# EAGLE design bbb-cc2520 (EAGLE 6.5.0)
AUTHOR: Neal Jackson; REV: D; TITLE: GAP

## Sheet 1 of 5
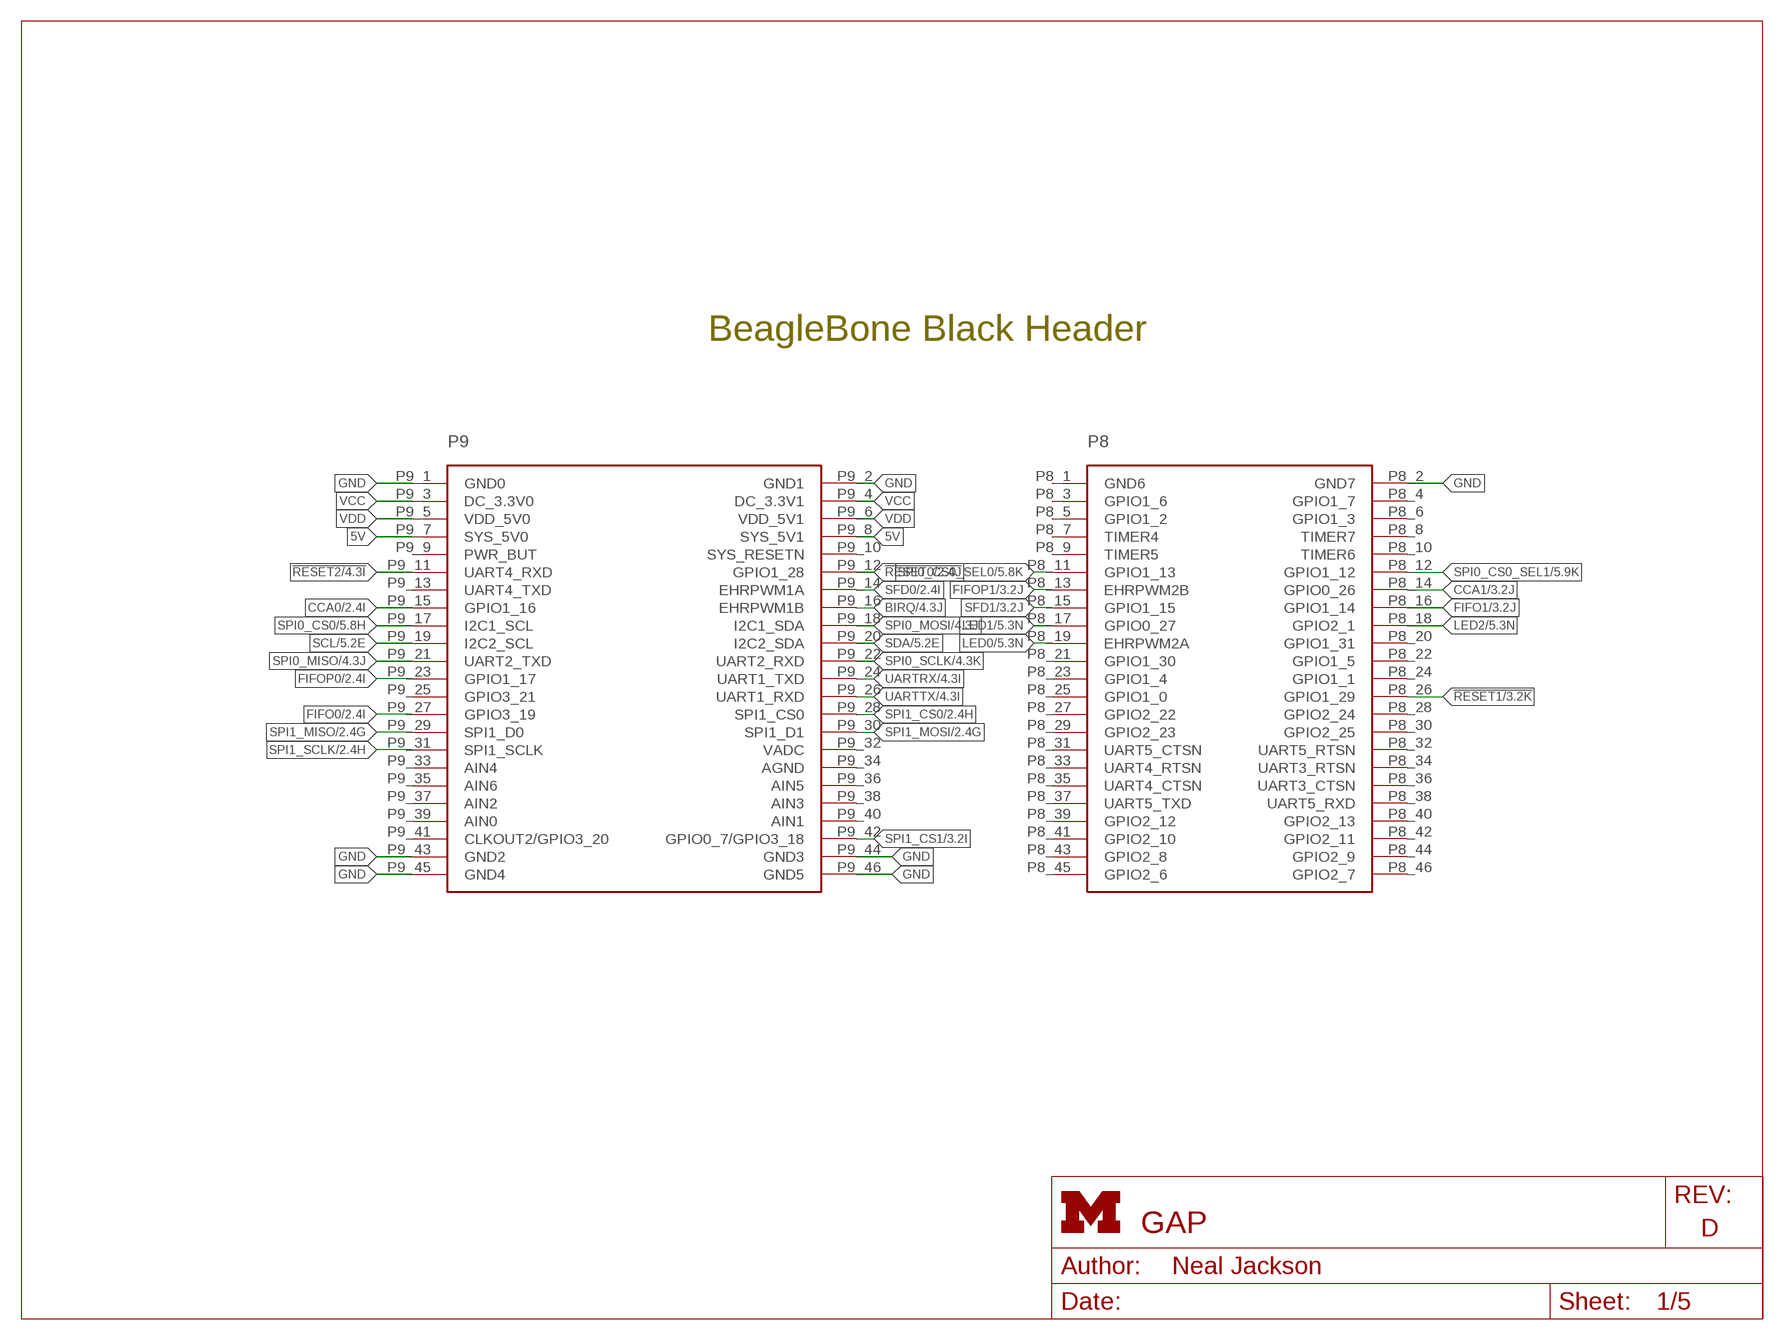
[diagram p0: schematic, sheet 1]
FRAME1 (LETTER_L): HEIGHT: 8.5in; WIDTH: 11in

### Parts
P9/P8  BBB_HEADERS  [BBB_HEADERS]

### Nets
5V: P9/P8.P9_7(SYS_5V0) P9/P8.P9_8(SYS_5V1)
!RESET0: P9/P8.P9_12(GPIO1_28) ; also sheet 2
!RESET1: P9/P8.P8_26(GPIO1_29) ; also sheet 3
!RESET2: P9/P8.P9_11(UART4_RXD) ; also sheet 4
BIRQ: P9/P8.P9_16(EHRPWM1B) ; also sheet 4
CCA0: P9/P8.P9_15(GPIO1_16) ; also sheet 2
CCA1: P9/P8.P8_14(GPIO0_26) ; also sheet 3
FIFO0: P9/P8.P9_27(GPIO3_19) ; also sheet 2
FIFO1: P9/P8.P8_16(GPIO1_14) ; also sheet 3
FIFOP0: P9/P8.P9_23(GPIO1_17) ; also sheet 2
FIFOP1: P9/P8.P8_13(EHRPWM2B) ; also sheet 3
GND: P9/P8.P8_2(GND7) P9/P8.P9_1(GND0) P9/P8.P9_2(GND1) P9/P8.P9_43(GND2) P9/P8.P9_44(GND3) P9/P8.P9_45(GND4) P9/P8.P9_46(GND5) ; also sheet 2,3,4,5
LED0: P9/P8.P8_19(EHRPWM2A) ; also sheet 5
LED1: P9/P8.P8_17(GPIO0_27) ; also sheet 5
LED2: P9/P8.P8_18(GPIO2_1) ; also sheet 5
SCL: P9/P8.P9_19(I2C2_SCL) ; also sheet 5
SDA: P9/P8.P9_20(I2C2_SDA) ; also sheet 5
SFD0: P9/P8.P9_14(EHRPWM1A) ; also sheet 2
SFD1: P9/P8.P8_15(GPIO1_15) ; also sheet 3
SPI0_CS0: P9/P8.P9_17(I2C1_SCL) ; also sheet 5
SPI0_CS0_SEL0: P9/P8.P8_11(GPIO1_13) ; also sheet 5
SPI0_CS0_SEL1: P9/P8.P8_12(GPIO1_12) ; also sheet 5
SPI0_MISO: P9/P8.P9_21(UART2_TXD) ; also sheet 4
SPI0_MOSI: P9/P8.P9_18(I2C1_SDA) ; also sheet 4
SPI0_SCLK: P9/P8.P9_22(UART2_RXD) ; also sheet 4
SPI1_CS0: P9/P8.P9_28(SPI1_CS0) ; also sheet 2
SPI1_CS1: P9/P8.P9_42(GPIO0_7/GPIO3_18) ; also sheet 3
SPI1_MISO: P9/P8.P9_29(SPI1_D0) ; also sheet 2,3
SPI1_MOSI: P9/P8.P9_30(SPI1_D1) ; also sheet 2,3
SPI1_SCLK: P9/P8.P9_31(SPI1_SCLK) ; also sheet 2,3
UARTRX: P9/P8.P9_24(UART1_TXD) ; also sheet 4
UARTTX: P9/P8.P9_26(UART1_RXD) ; also sheet 4
VCC: P9/P8.P9_3(DC_3.3V0) P9/P8.P9_4(DC_3.3V1) ; also sheet 2,3,4,5
VDD: P9/P8.P9_5(VDD_5V0) P9/P8.P9_6(VDD_5V1)
Unconnected: P9/P8.P8_1(GND6) P9/P8.P8_3(GPIO1_6) P9/P8.P8_4(GPIO1_7) P9/P8.P8_5(GPIO1_2) P9/P8.P8_6(GPIO1_3) P9/P8.P8_7(TIMER4) P9/P8.P8_8(TIMER7) P9/P8.P8_9(TIMER5) P9/P8.P8_10(TIMER6) P9/P8.P8_20(GPIO1_31) P9/P8.P8_21(GPIO1_30) P9/P8.P8_22(GPIO1_5) P9/P8.P8_23(GPIO1_4) P9/P8.P8_24(GPIO1_1) P9/P8.P8_25(GPIO1_0) P9/P8.P8_27(GPIO2_22) P9/P8.P8_28(GPIO2_24) P9/P8.P8_29(GPIO2_23) P9/P8.P8_30(GPIO2_25) P9/P8.P8_31(UART5_CTSN) P9/P8.P8_32(UART5_RTSN) P9/P8.P8_33(UART4_RTSN) P9/P8.P8_34(UART3_RTSN) P9/P8.P8_35(UART4_CTSN) P9/P8.P8_36(UART3_CTSN) P9/P8.P8_37(UART5_TXD) P9/P8.P8_38(UART5_RXD) P9/P8.P8_39(GPIO2_12) P9/P8.P8_40(GPIO2_13) P9/P8.P8_41(GPIO2_10) P9/P8.P8_42(GPIO2_11) P9/P8.P8_43(GPIO2_8) P9/P8.P8_44(GPIO2_9) P9/P8.P8_45(GPIO2_6) P9/P8.P8_46(GPIO2_7) P9/P8.P9_9(PWR_BUT) P9/P8.P9_10(SYS_RESETN) P9/P8.P9_13(UART4_TXD) P9/P8.P9_25(GPIO3_21) P9/P8.P9_32(VADC) P9/P8.P9_33(AIN4) P9/P8.P9_34(AGND) P9/P8.P9_35(AIN6) P9/P8.P9_36(AIN5) P9/P8.P9_37(AIN2) P9/P8.P9_38(AIN3) P9/P8.P9_39(AIN0) P9/P8.P9_40(AIN1) P9/P8.P9_41(CLKOUT2/GPIO3_20)

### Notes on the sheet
- BeagleBone Black Header

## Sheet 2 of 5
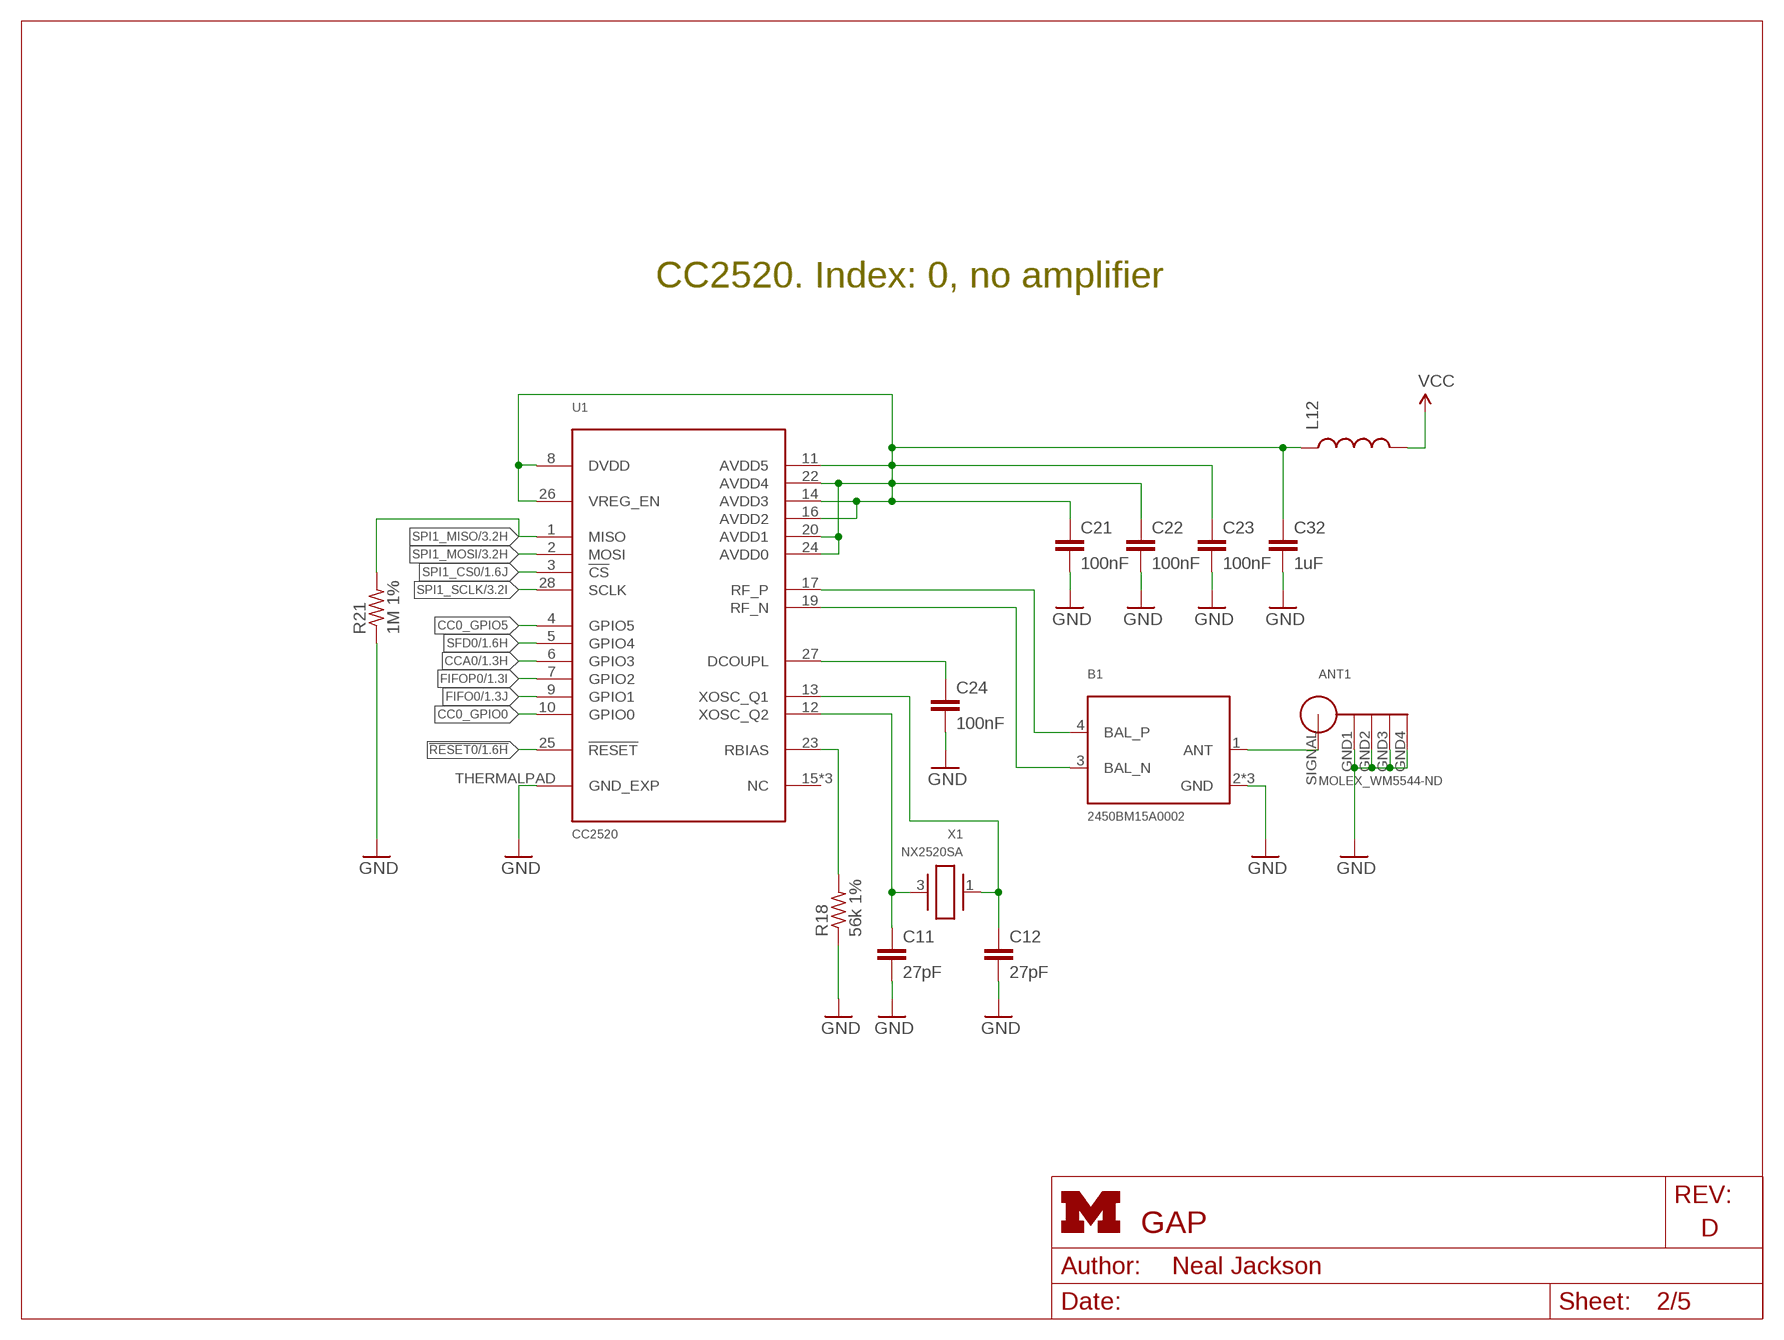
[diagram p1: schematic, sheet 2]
FRAME6 (LETTER_L): HEIGHT: 8.5in; WIDTH: 11in

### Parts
ANT1  MOLEX_WM5544-ND  [MOLEX_WM5544-ND]
B1  2450BM15A0002  [2450BM]
C11  27pF  C-EUC0402  [C0402]
C12  27pF  C-EUC0402  [C0402]
C21  100nF  C-EUC0402  [C0402]
C22  100nF  C-EUC0402  [C0402]
C23  100nF  C-EUC0402  [C0402]
C24  100nF  C-EUC0402  [C0402]
C32  1uF  C-EUC0603  [C0603]
L12  INDUCTOR0603  [0603]
R18  56k 1%  R-US_R0402  [R0402]
R21  1M 1%  R-US_R0402  [R0402]
U1  CC2520  [S-PVQFN-N28]
X1  NX2520SA  [NX2520SA]

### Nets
!RESET0: U1.25(!RESET) ; also sheet 1
CC0_GPIO0: U1.10(GPIO0)
CC0_GPIO5: U1.4(GPIO5)
CCA0: U1.6(GPIO3) ; also sheet 1
FIFO0: U1.9(GPIO1) ; also sheet 1
FIFOP0: U1.7(GPIO2) ; also sheet 1
GND: ANT1.GND1 ANT1.GND2 ANT1.GND3 ANT1.GND4 B1.2(GND) B1.5(GND) B1.6(GND) C11.2 C12.2 C21.2 C22.2 C23.2 C24.2 C32.2 R18.1 R21.1 U1.THERMALPAD(GND_EXP) ; also sheet 1,3,4,5
N$5: C21.1 C22.1 C23.1 C32.1 L12.1 U1.8(DVDD) U1.11(AVDD5) U1.14(AVDD3) U1.16(AVDD2) U1.20(AVDD1) U1.22(AVDD4) U1.24(AVDD0) U1.26(VREG_EN)
N$7: ANT1.SIGNAL B1.1(ANT)
N$11: C12.1 U1.13(XOSC_Q1) X1.1
N$12: C24.1 U1.27(DCOUPL)
N$13: C11.1 U1.12(XOSC_Q2) X1.3
N$14: R18.2 U1.23(RBIAS)
RF_N: B1.3(BAL_N) U1.19(RF_N)
RF_P: B1.4(BAL_P) U1.17(RF_P)
SFD0: U1.5(GPIO4) ; also sheet 1
SPI1_CS0: U1.3(!CS) ; also sheet 1
SPI1_MISO: R21.2 U1.1(MISO) ; also sheet 1,3
SPI1_MOSI: U1.2(MOSI) ; also sheet 1,3
SPI1_SCLK: U1.28(SCLK) ; also sheet 1,3
VCC: L12.2 ; also sheet 1,3,4,5
Unconnected: U1.15(NC) U1.18(NC) U1.21(NC)

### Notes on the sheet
- CC2520. Index: 0, no amplifier

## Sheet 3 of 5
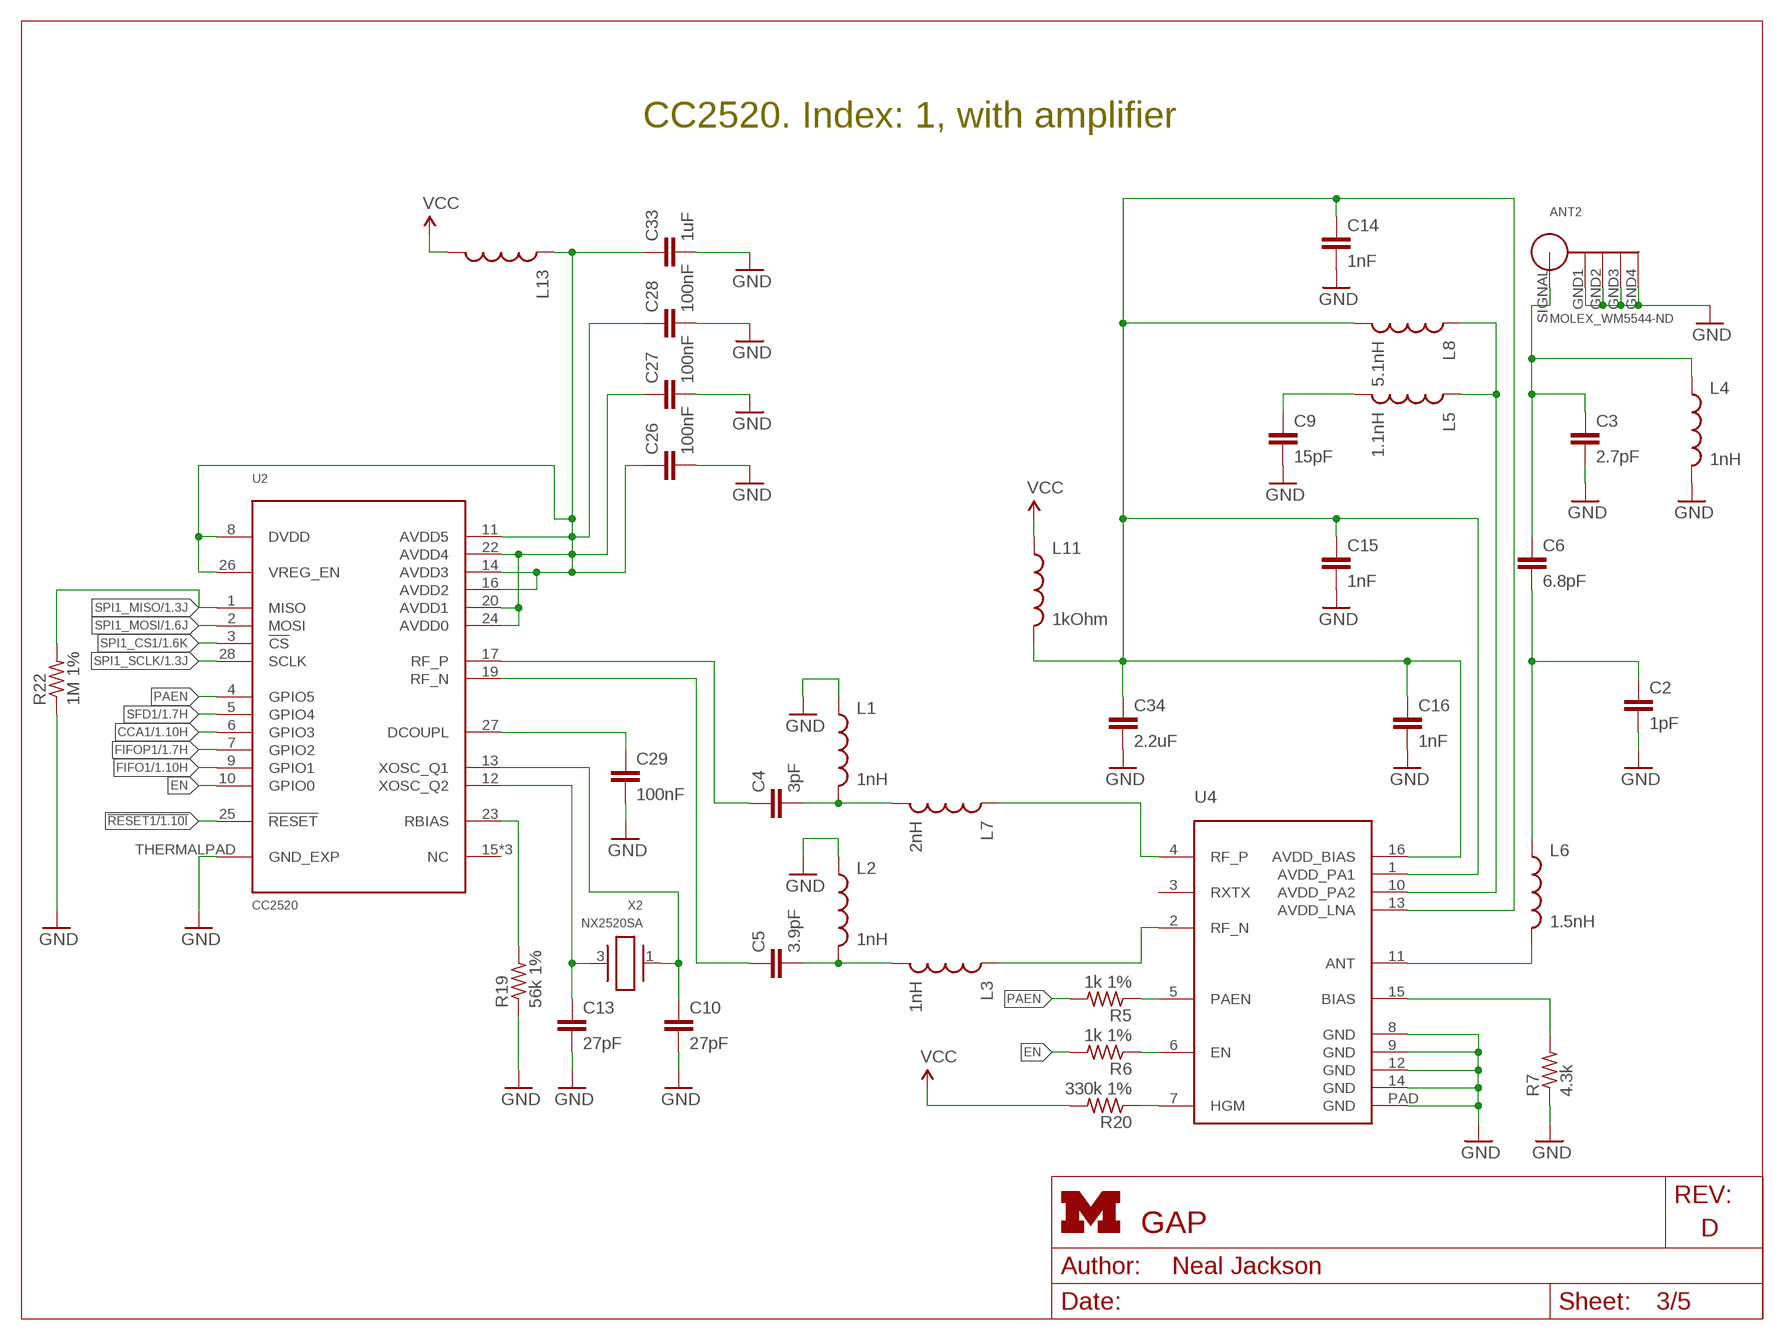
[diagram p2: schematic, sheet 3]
FRAME3 (LETTER_L): HEIGHT: 8.5in; WIDTH: 11in

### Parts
ANT2  MOLEX_WM5544-ND  [MOLEX_WM5544-ND]
C2  1pF  C-EUC0402  [C0402]
C3  2.7pF  C-EUC0402  [C0402]
C4  3pF  C-EUC0402  [C0402]
C5  3.9pF  C-EUC0402  [C0402]
C6  6.8pF  C-EUC0402  [C0402]
C9  15pF  C-EUC0402  [C0402]
C10  27pF  C-EUC0402  [C0402]
C13  27pF  C-EUC0402  [C0402]
C14  1nF  C-EUC0402  [C0402]
C15  1nF  C-EUC0402  [C0402]
C16  1nF  C-EUC0402  [C0402]
C26  100nF  C-EUC0402  [C0402]
C27  100nF  C-EUC0402  [C0402]
C28  100nF  C-EUC0402  [C0402]
C29  100nF  C-EUC0402  [C0402]
C33  1uF  C-EUC0603  [C0603]
C34  2.2uF  C-EUC0402  [C0402]
L1  1nH  INDUCTOR0402  [C0402]
L2  1nH  INDUCTOR0402  [C0402]
L3  1nH  INDUCTOR0402  [C0402]
L4  1nH  INDUCTOR0402  [C0402]
L5  1.1nH  INDUCTOR0402  [C0402]
L6  1.5nH  INDUCTOR0402  [C0402]
L7  2nH  INDUCTOR0402  [C0402]
L8  5.1nH  INDUCTOR0402  [C0402]
L11  1kOhm  INDUCTOR0402  [C0402]
L13  INDUCTOR0603  [0603]
R5  1k 1%  R-US_R0402  [R0402]
R6  1k 1%  R-US_R0402  [R0402]
R7  4.3k  R-US_R0402  [R0402]
R19  56k 1%  R-US_R0402  [R0402]
R20  330k 1%  R-US_R0402  [R0402]
R22  1M 1%  R-US_R0402  [R0402]
U2  CC2520  [S-PVQFN-N28]
U4  CC2591  [PVQFN-16]
X2  NX2520SA  [NX2520SA]

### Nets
!RESET1: U2.25(!RESET) ; also sheet 1
CCA1: U2.6(GPIO3) ; also sheet 1
EN: R6.2 U2.10(GPIO0)
FIFO1: U2.9(GPIO1) ; also sheet 1
FIFOP1: U2.7(GPIO2) ; also sheet 1
GND: ANT2.GND1 ANT2.GND2 ANT2.GND3 ANT2.GND4 C2.2 C3.2 C9.2 C10.2 C13.2 C14.2 C15.2 C16.2 C26.2 C27.2 C28.2 C29.2 C33.2 C34.2 L1.1 L2.1 L4.2 R7.1 R19.1 R22.1 U2.THERMALPAD(GND_EXP) U4.8(GND) U4.9(GND) U4.12(GND) U4.14(GND) U4.PAD(GND) ; also sheet 1,2,4,5
N$44: L7.1 U4.4(RF_P)
N$45: L3.1 U4.2(RF_N)
N$46: C5.2 L2.2 L3.2
N$47: C4.2 L1.2 L7.2
N$48: L5.1 L8.1 U4.10(AVDD_PA2)
N$49: C14.1 C15.1 C16.1 C34.1 L8.2 L11.2 U4.1(AVDD_PA1) U4.13(AVDD_LNA) U4.16(AVDD_BIAS)
N$50: C9.1 L5.2
N$51: L6.2 U4.11(ANT)
N$52: ANT2.SIGNAL C3.1 C6.1 L4.1
N$53: C2.1 C6.2 L6.1
N$54: R7.2 U4.15(BIAS)
N$55: R5.1 U4.5(PAEN)
N$56: R6.1 U4.6(EN)
N$57: C26.1 C27.1 C28.1 C33.1 L13.1 U2.8(DVDD) U2.11(AVDD5) U2.14(AVDD3) U2.16(AVDD2) U2.20(AVDD1) U2.22(AVDD4) U2.24(AVDD0) U2.26(VREG_EN)
N$58: C29.1 U2.27(DCOUPL)
N$59: C10.1 U2.13(XOSC_Q1) X2.1
N$60: C13.1 U2.12(XOSC_Q2) X2.3
N$61: R19.2 U2.23(RBIAS)
N$62: R20.1 U4.7(HGM)
PAEN: R5.2 U2.4(GPIO5)
RF_N2: C5.1 U2.19(RF_N)
RF_P2: C4.1 U2.17(RF_P)
SFD1: U2.5(GPIO4) ; also sheet 1
SPI1_CS1: U2.3(!CS) ; also sheet 1
SPI1_MISO: R22.2 U2.1(MISO) ; also sheet 1,2
SPI1_MOSI: U2.2(MOSI) ; also sheet 1,2
SPI1_SCLK: U2.28(SCLK) ; also sheet 1,2
VCC: L11.1 L13.2 R20.2 ; also sheet 1,2,4,5
Unconnected: U2.15(NC) U2.18(NC) U2.21(NC) U4.3(RXTX)

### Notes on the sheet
- CC2520. Index: 1, with amplifier

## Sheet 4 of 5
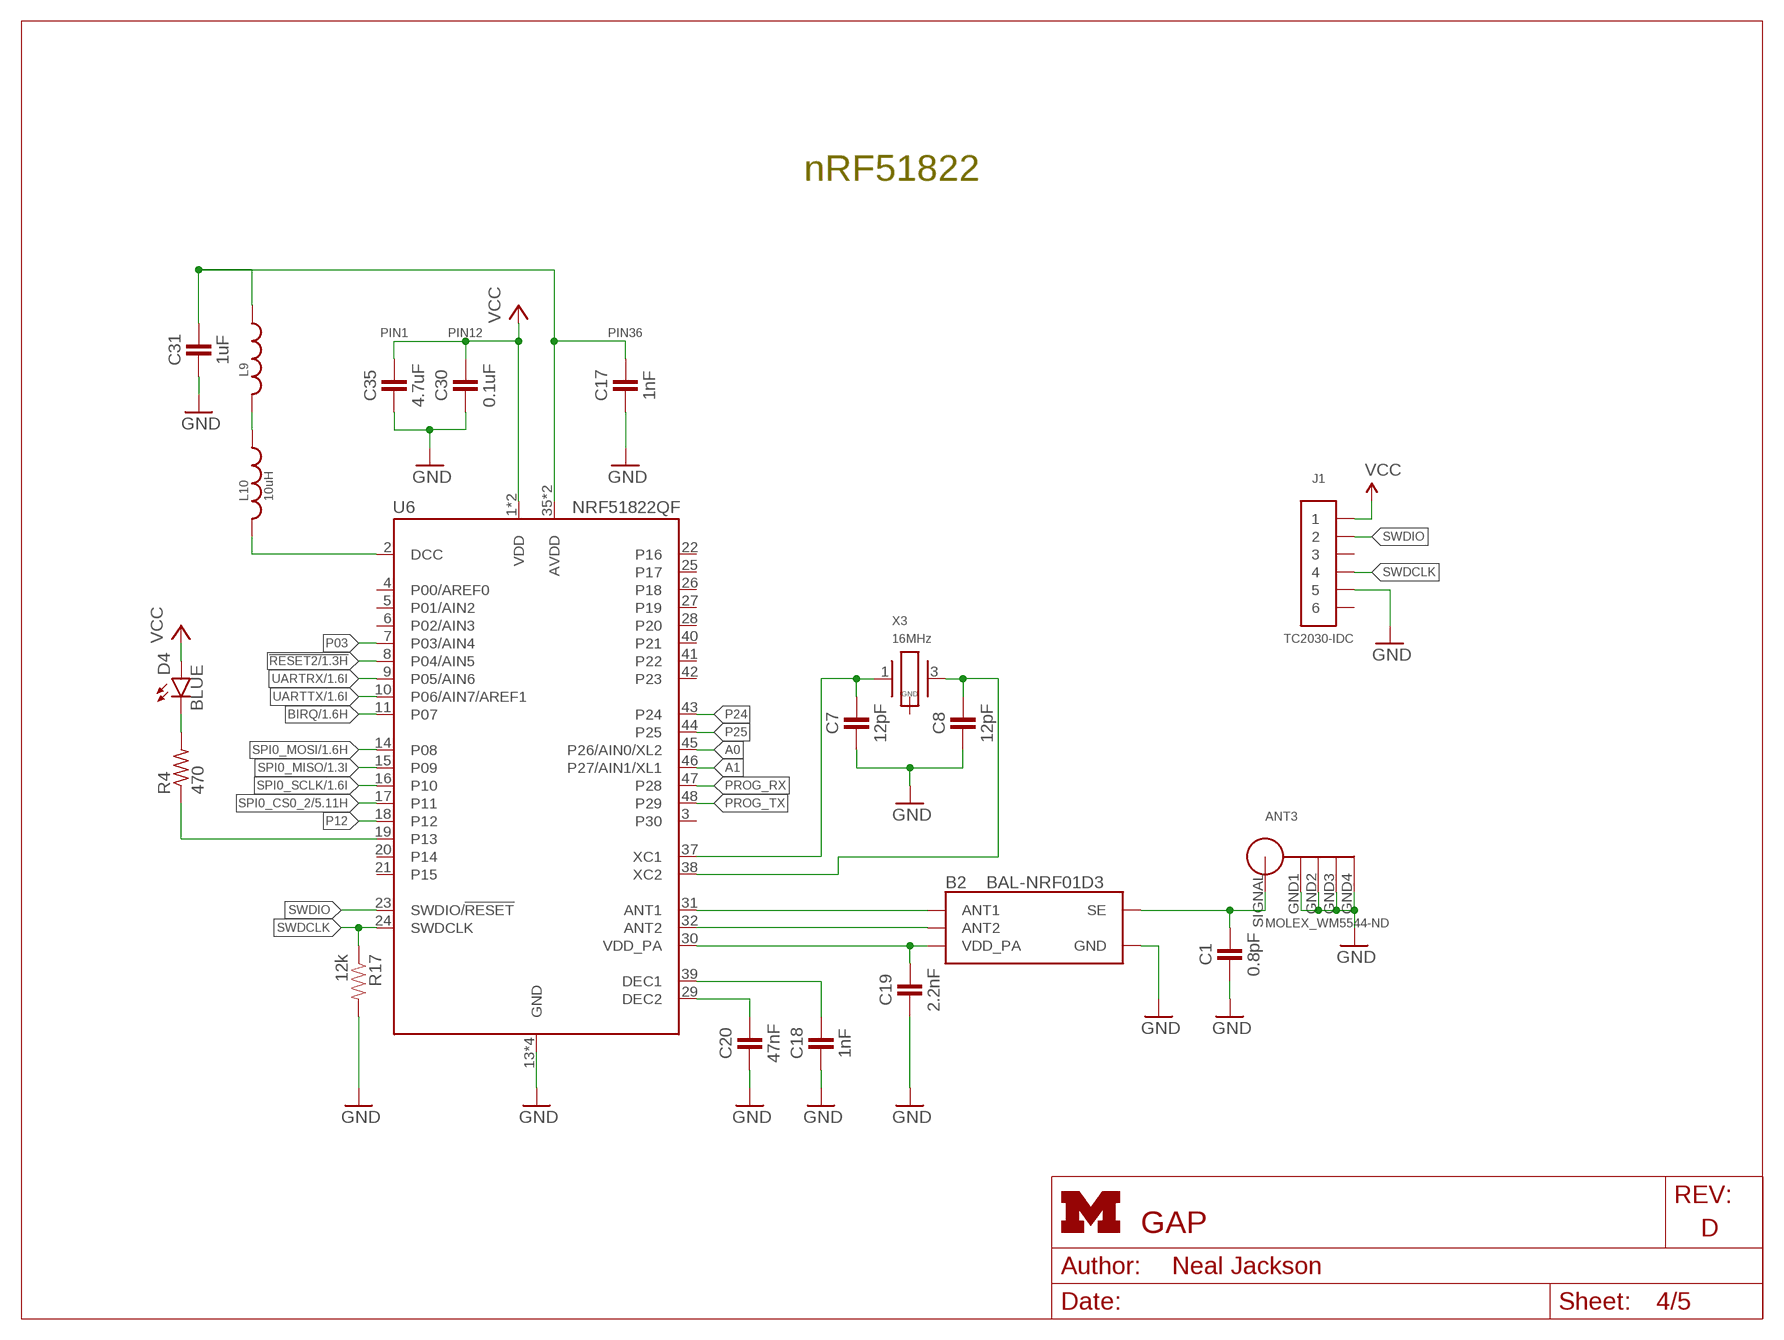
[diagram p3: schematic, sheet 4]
FRAME2 (LETTER_L): HEIGHT: 8.5in; WIDTH: 11in

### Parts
ANT3  MOLEX_WM5544-ND  [MOLEX_WM5544-ND]
B2  BAL-NRF01D3  [BAL-NRF01D3]
C1  0.8pF  CAPACITOR  [0402_CAP]
C7  12pF  CAPACITOR  [0402_CAP]
C8  12pF  CAPACITOR  [0402_CAP]
C17  1nF  CAPACITOR  [0402_CAP]
C18  1nF  CAPACITOR  [0402_CAP]
C19  2.2nF  CAPACITOR  [0402_CAP]
C20  47nF  CAPACITOR  [0402_CAP]
C30  0.1uF  CAPACITOR  [0402_CAP]
C31  1uF  CAPACITOR  [0402_CAP]
C35  4.7uF  CAPACITOR  [0402_CAP]
D4  BLUE  LED0603  [LED-0603]
J1  TC2030-IDC  [TC2030-IDC]
L9  INDUCTOR0402  [0402_CAP]
L10  10uH  INDUCTOR0603  [0603_CAP]
R4  470  R-US_R0402  [R0402]
R17  12k  RESISTOR  [0603-RES]
U6  NRF51822QF  [QFN-48-6MM]
X3  16MHz  TXC-8Y  [TXC-8Y]

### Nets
!RESET2: U6.8(P04/AIN5) ; also sheet 1
A0: U6.45(P26/AIN0/XL2)
A1: U6.46(P27/AIN1/XL1)
AVDD: C17.1 C31.1 L9.1 U6.35(AVDD) U6.36(AVDD)
BIRQ: U6.11(P07) ; also sheet 1
DCC: L10.2 U6.2(DCC)
GND: ANT3.GND1 ANT3.GND2 ANT3.GND3 ANT3.GND4 B2.GND C1.2 C7.2 C8.2 C17.2 C18.2 C19.2 C20.2 C30.2 C31.2 C35.2 J1.5 R17.2 U6.13(GND) U6.33(GND) U6.34(GND) U6.GND ; also sheet 1,2,3,5
N$36: B2.ANT1 U6.31(ANT1)
N$37: B2.ANT2 U6.32(ANT2)
N$38: ANT3.SIGNAL B2.SE C1.1
N$39: L9.2 L10.1
N$40: C7.1 U6.37(XC1) X3.1
N$41: C8.1 U6.38(XC2) X3.3
N$42: C18.1 U6.39(DEC1)
N$43: C20.1 U6.29(DEC2)
N$63: D4.C R4.2
N$64: R4.1 U6.19(P13)
P03: U6.7(P03/AIN4)
P12: U6.18(P12)
P24: U6.43(P24)
P25: U6.44(P25)
PROG_RX: U6.47(P28)
PROG_TX: U6.48(P29)
SPI0_CS0_2: U6.17(P11) ; also sheet 5
SPI0_MISO: U6.15(P09) ; also sheet 1
SPI0_MOSI: U6.14(P08) ; also sheet 1
SPI0_SCLK: U6.16(P10) ; also sheet 1
SWDCLK: J1.4 R17.1 U6.24(SWDCLK)
SWDIO: J1.2 U6.23(SWDIO/!RESET)
UARTRX: U6.9(P05/AIN6) ; also sheet 1
UARTTX: U6.10(P06/AIN7/AREF1) ; also sheet 1
VCC: C30.1 C35.1 D4.A J1.1 U6.1(VDD) U6.12(VDD) ; also sheet 1,2,3,5
VDD_PA: B2.VCC(VDD_PA) C19.1 U6.30(VDD_PA)
Unconnected: J1.3 J1.6 U6.3(P30) U6.4(P00/AREF0) U6.5(P01/AIN2) U6.6(P02/AIN3) U6.20(P14) U6.21(P15) U6.22(P16) U6.25(P17) U6.26(P18) U6.27(P19) U6.28(P20) U6.40(P21) U6.41(P22) U6.42(P23) X3.2(GND) X3.4(GND)

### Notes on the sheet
- nRF51822
- PIN1 | PIN12 | PIN36

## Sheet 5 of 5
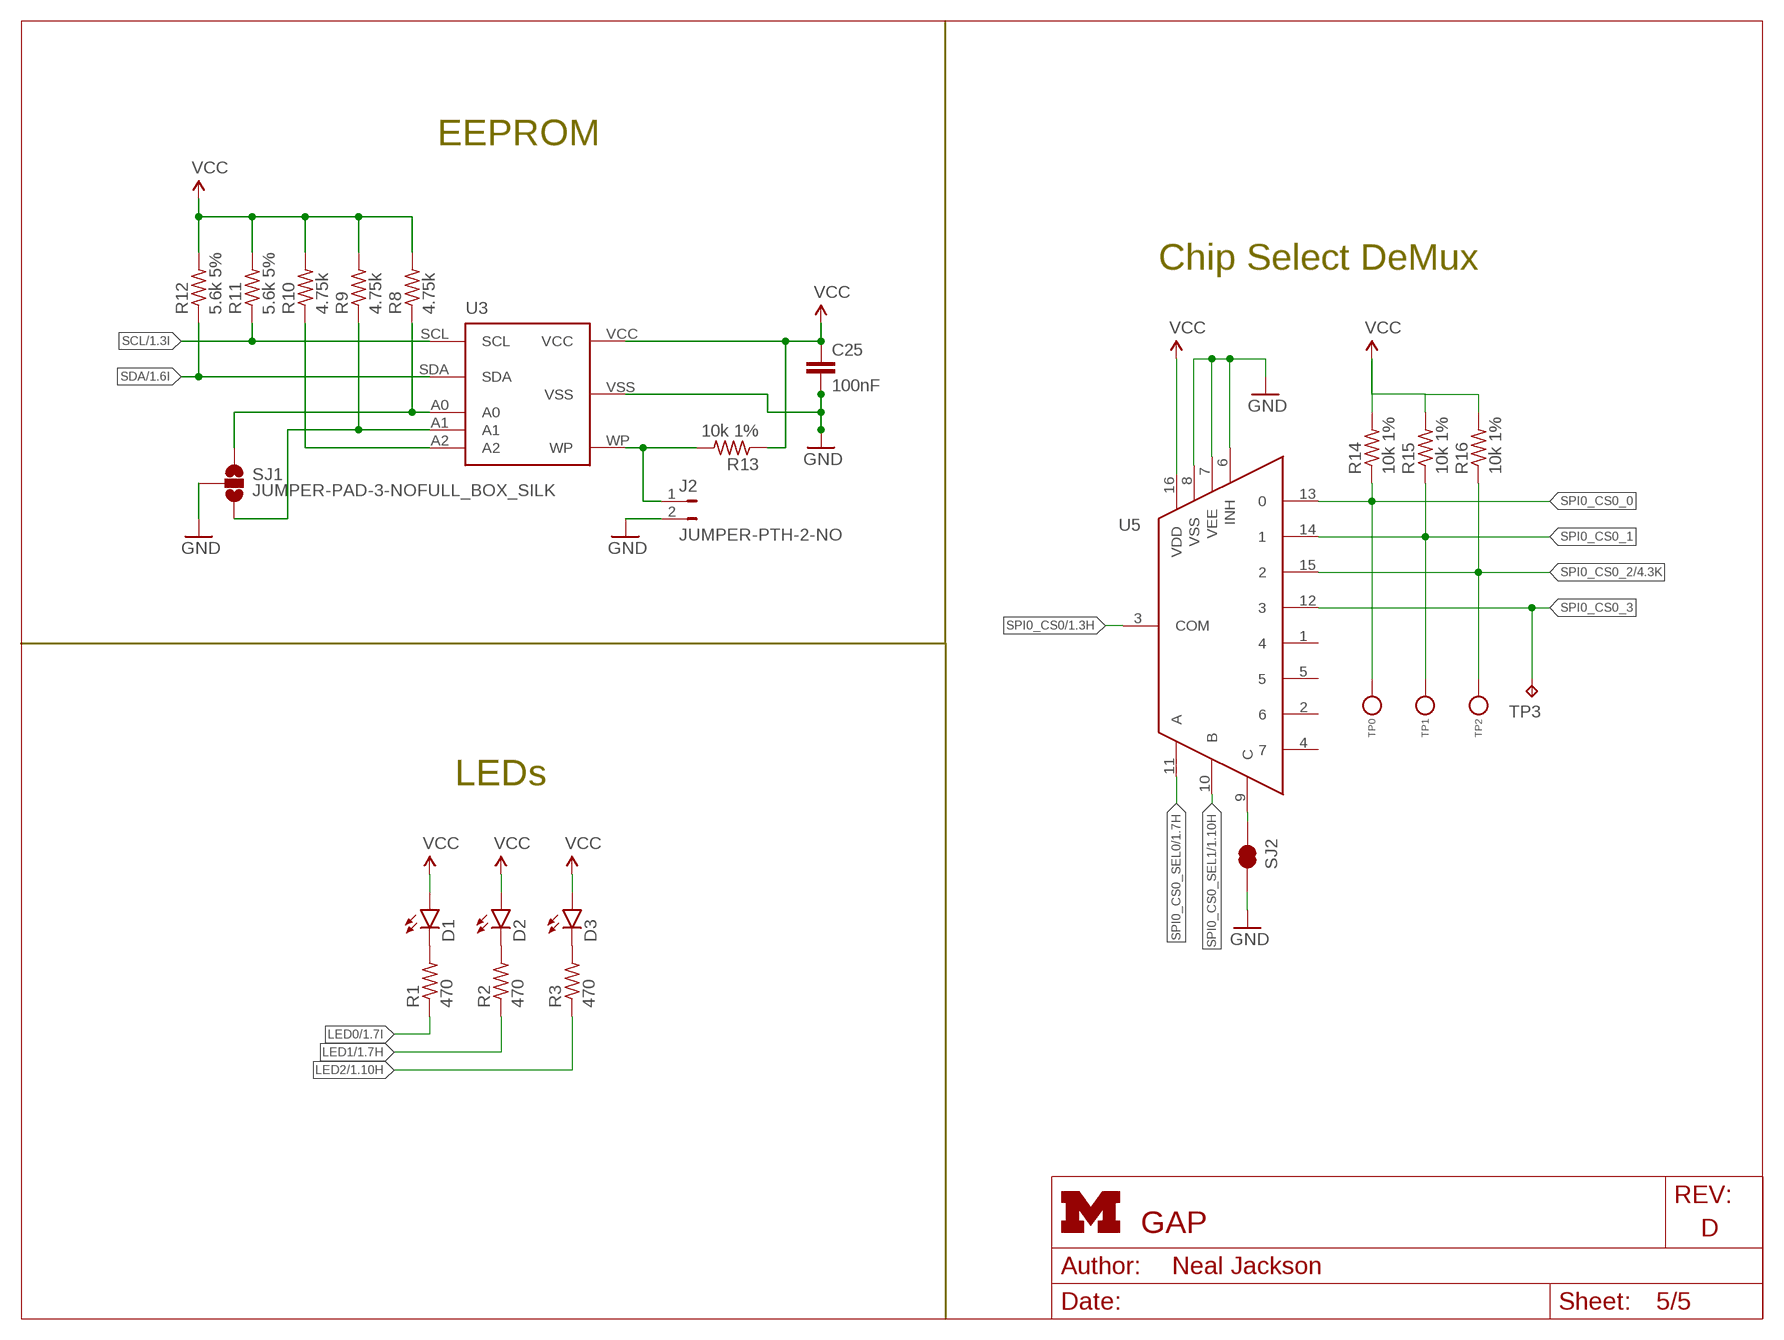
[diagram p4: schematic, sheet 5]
FRAME4 (LETTER_L): HEIGHT: 8.5in; WIDTH: 11in

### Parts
C25  100nF  C-EUC0402  [C0402]
D1  LED0603  [LED-0603]
D2  LED0603  [LED-0603]
D3  LED0603  [LED-0603]
J2  JUMPER-PTH-2-NO  [PTH-JUMPER-2-NO_NO_SILK]
R1  470  R-US_R0402  [R0402]
R2  470  R-US_R0402  [R0402]
R3  470  R-US_R0402  [R0402]
R8  4.75k  R-US_R0402  [R0402]
R9  4.75k  R-US_R0402  [R0402]
R10  4.75k  R-US_R0402  [R0402]
R11  5.6k 5%  R-US_R0402  [R0402]
R12  5.6k 5%  R-US_R0402  [R0402]
R13  10k 1%  R-US_R0402  [R0402]
R14  10k 1%  R-US_R0402  [R0402]
R15  10k 1%  R-US_R0402  [R0402]
R16  10k 1%  R-US_R0402  [R0402]
SJ1  JUMPER-PAD-3-NOFULL_BOX_SILK  [PAD-JUMPER-3-NO_YES_SILK_FULL_BOX]
SJ2  JUMPER-PAD-2-NC_BY_TRACE  [PAD-JUMPER-2-NC_BY_TRACE_YES_SILK]
TP0  TEST_POINT_0.040IN  [TESTPOINT_0.040IN]
TP1  TEST_POINT_0.040IN  [TESTPOINT_0.040IN]
TP2  TEST_POINT_0.040IN  [TESTPOINT_0.040IN]
TP3  TPTP14SQ  [TP14SQ]
U3  CAT24C256WI-GT3  [CAT24C256WI-GT3]
U5  CD4051B-53B  [TSSOP16]

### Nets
GND: C25.2 J2.2 SJ1.2 SJ2.2 U3.VSS U5.6(INH) U5.7(VEE) U5.8(VSS) ; also sheet 1,2,3,4
LED0: R1.1 ; also sheet 1
LED1: R2.1 ; also sheet 1
LED2: R3.1 ; also sheet 1
N$1: D1.C R1.2
N$2: D2.C R2.2
N$3: D3.C R3.2
N$29: R8.1 SJ1.1 U3.A0
N$30: R9.1 SJ1.3 U3.A1
N$31: J2.1 R13.2 U3.WP
N$32: R10.1 U3.A2
N$65: SJ2.1 U5.9(C)
SCL: R11.1 U3.SCL ; also sheet 1
SDA: R12.1 U3.SDA ; also sheet 1
SPI0_CS0: U5.3(COM) ; also sheet 1
SPI0_CS0_0: R14.1 TP0.TESTPOINT U5.13
SPI0_CS0_1: R15.1 TP1.TESTPOINT U5.14
SPI0_CS0_2: R16.1 TP2.TESTPOINT U5.15 ; also sheet 4
SPI0_CS0_3: TP3.TP U5.12
SPI0_CS0_SEL0: U5.11(A) ; also sheet 1
SPI0_CS0_SEL1: U5.10(B) ; also sheet 1
VCC: C25.1 D1.A D2.A D3.A R8.2 R9.2 R10.2 R11.2 R12.2 R13.1 R14.2 R15.2 R16.2 U3.VCC U5.16(VDD) ; also sheet 1,2,3,4
Unconnected: U5.1 U5.2 U5.4 U5.5

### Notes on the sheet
- EEPROM
- Chip Select DeMux
- LEDs

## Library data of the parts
ANT1-ANT3 = connector:MOLEX_WM5544-ND: Through-hole SMA Antenna; DIGIKEY: WM5544-ND
B1 = rpi-cc2520:2450BM15A0002: BALUN JTI MATCHED ZIGBEE; DIGIKEY: 712-1536-1-ND
B2 = chips:BAL-NRF01D3: 50 ohm nominal input / conjugate match balun to nRF51422-QFAA, nRF24LE1, nRF51822-QFAA/AB, with integrated harmonic filter; DIGIKEY: 497-13637-1-ND; MOUSER: 511-BAL-NRF01D3
C1 C19 = passives:CAPACITOR: 0402 Capacitor; DIGIKEY: 490-5419-1-ND
C2-C6 C9 C14-C16 C21-C29 C34 = rcl:C-EU: CAPACITOR, European symbol; DIGIKEY: 490-1318-1-ND
C7 C8 = passives:CAPACITOR: 0402 Capacitor; DIGIKEY: 490-6197-1-ND
C10-C13 = rcl:C-EU: CAPACITOR, European symbol; DIGIKEY: 490-5869-1-ND
C17 C18 = passives:CAPACITOR: 0402 Capacitor; DIGIKEY: 490-1303-1-ND
C20 = passives:CAPACITOR: 0402 Capacitor; DIGIKEY: 445-1264-1-ND
C30 = passives:CAPACITOR: 0402 Capacitor; DIGIKEY: 445-4952-1-ND
C31 = passives:CAPACITOR: 0402 Capacitor; DIGIKEY: 1276-1513-1-ND
C32 C33 = rcl:C-EU: CAPACITOR, European symbol; DIGIKEY: 490-1550-1-ND
C35 = passives:CAPACITOR: 0402 Capacitor; DIGIKEY: 445-5947-1-ND
D1 = SparkFun-LED:LED: LEDs; DIGIKEY: 160-1834-1-ND
D2 = SparkFun-LED:LED: LEDs; DIGIKEY: 160-1835-1-ND
D3 = SparkFun-LED:LED: LEDs; DIGIKEY: 160-1837-1-ND
D4 = SparkFun-LED:LED: LEDs
J1 = connector:TC2030-IDC: The TC2030-IDC is our "Legged" 6-pin Plug-of-Nailstm Cable fitted with a 6-pin 0.1" pitch ribbon connector.; TAGCONNECT: TC2030-IDC
J2 = SparkFun-Passives:JUMPER-PTH-2-NO
L1-L8 L11 = SparkFun-Passives:INDUCTOR: Inductors
L9 = passives:INDUCTOR; DIGIKEY: 587-1521-1-ND
L10 = passives:INDUCTOR; DIGIKEY: 490-4025-1-ND
L12 L13 = SparkFun-Passives:INDUCTOR: Inductors; DIGIKEY: 490-1015-1-ND
P9/P8 = bbb-cc2520:BBB_HEADERS: Pin Header 2x23
R1-R4 = rcl:R-US_: RESISTOR, American symbol; DIGIKEY: RHM470JCT-ND
R5-R7 R18-R20 = rcl:R-US_: RESISTOR, American symbol; DIGIKEY: P56.0KLCT-ND
R8-R16 R21 R22 = rcl:R-US_: RESISTOR, American symbol; DIGIKEY: RHM1.00MCDCT-ND
R17 = passives:RESISTOR: Resistor; DIGIKEY: RHM12.0KCDCT-ND
SJ1 = SparkFun-Passives:JUMPER-PAD-3-NO
SJ2 = SparkFun-Passives:JUMPER-PAD-2-NC_BY_TRACE
TP0 TP1 TP2 = headers:TEST_POINT_0.040IN: 0.040in Test Point; DIGIKEY: 5001K-ND
TP3 = testpad:TP: Test pad
U1 U2 = chips:CC2520: 2.4 GHZ IEEE 802.15.4/ZIGBEE® RF TRANSCEIVER; DIGIKEY: 296-22996-1-ND
U3 = bbb-cc2520:CAT24C256: 256kb Serial CMOS EEPROM, organized as 32,768 words of 8 bits each
U4 = bbb-cc2520:CC2591
U5 = bbb-cc2520:CD4051B-53B: IC MUX/DEMUX 8x1 16TSSOP; DIGIKEY: 296-11993-1-ND
U6 = chips:NRF51822: Multiprotocol Bluetooth® 4.0 low energy/2.4 GHz RF SoC; DIGIKEY: 1490-1032-1-ND; MOUSER: 949-NRF51822-QFAB-R7
X1 X2 = rpi-cc2520:NX2520SA: CRYSTAL 32MHZ 10PF SMD; DIGIKEY: 644-1065-1-ND
X3 = crystals:TXC-8Y: 2mmx1.6mm SMD Crystal; DIGIKEY: 887-2003-1-ND

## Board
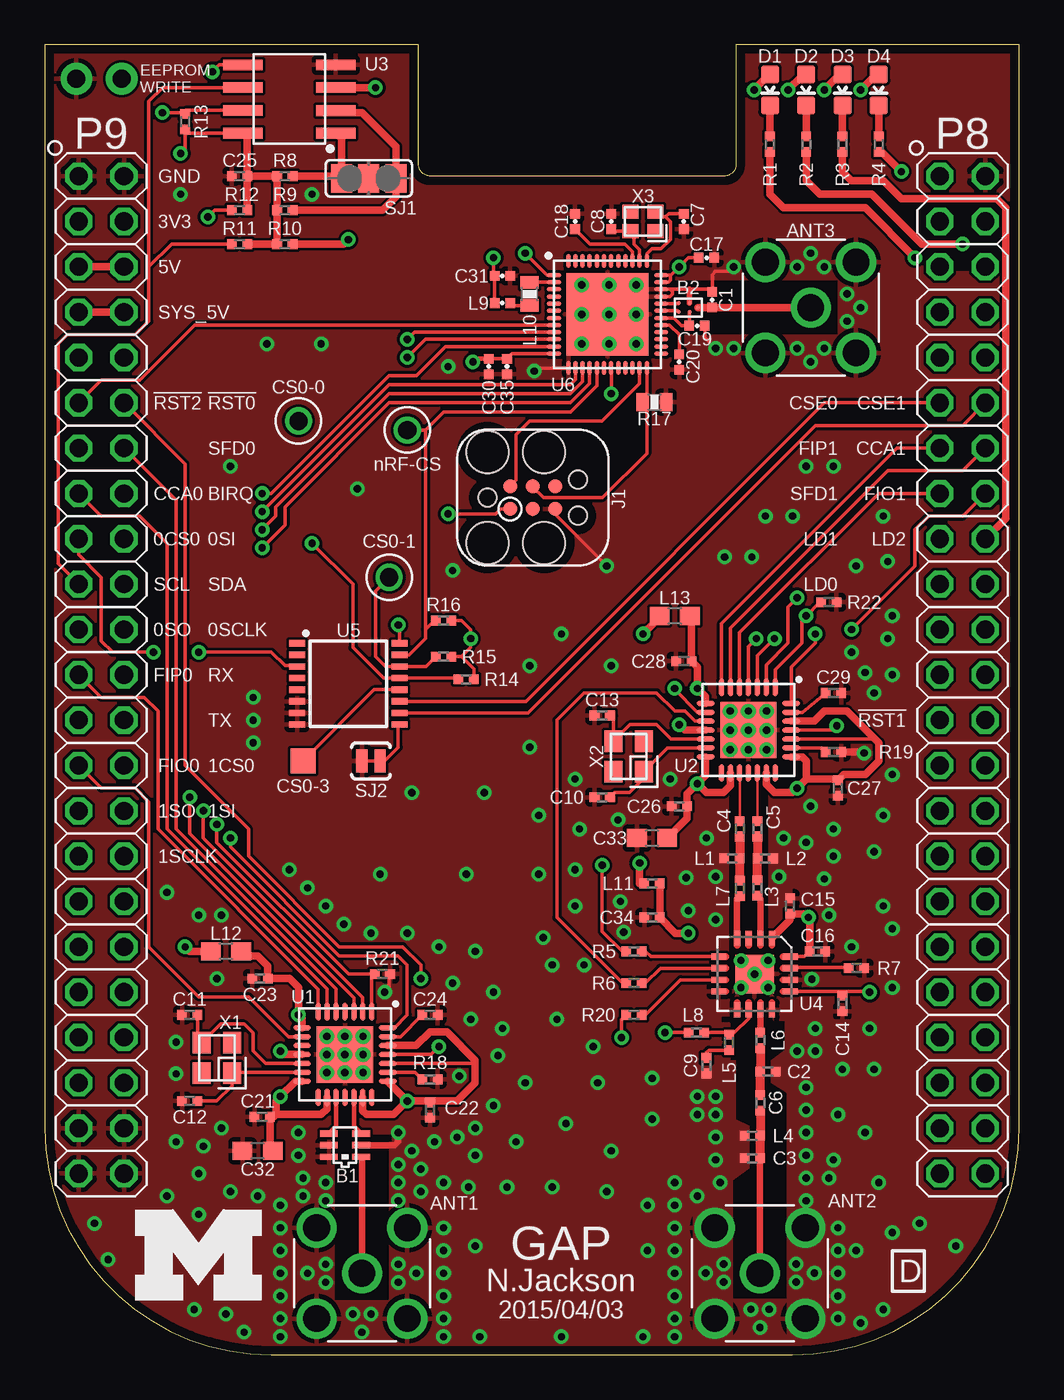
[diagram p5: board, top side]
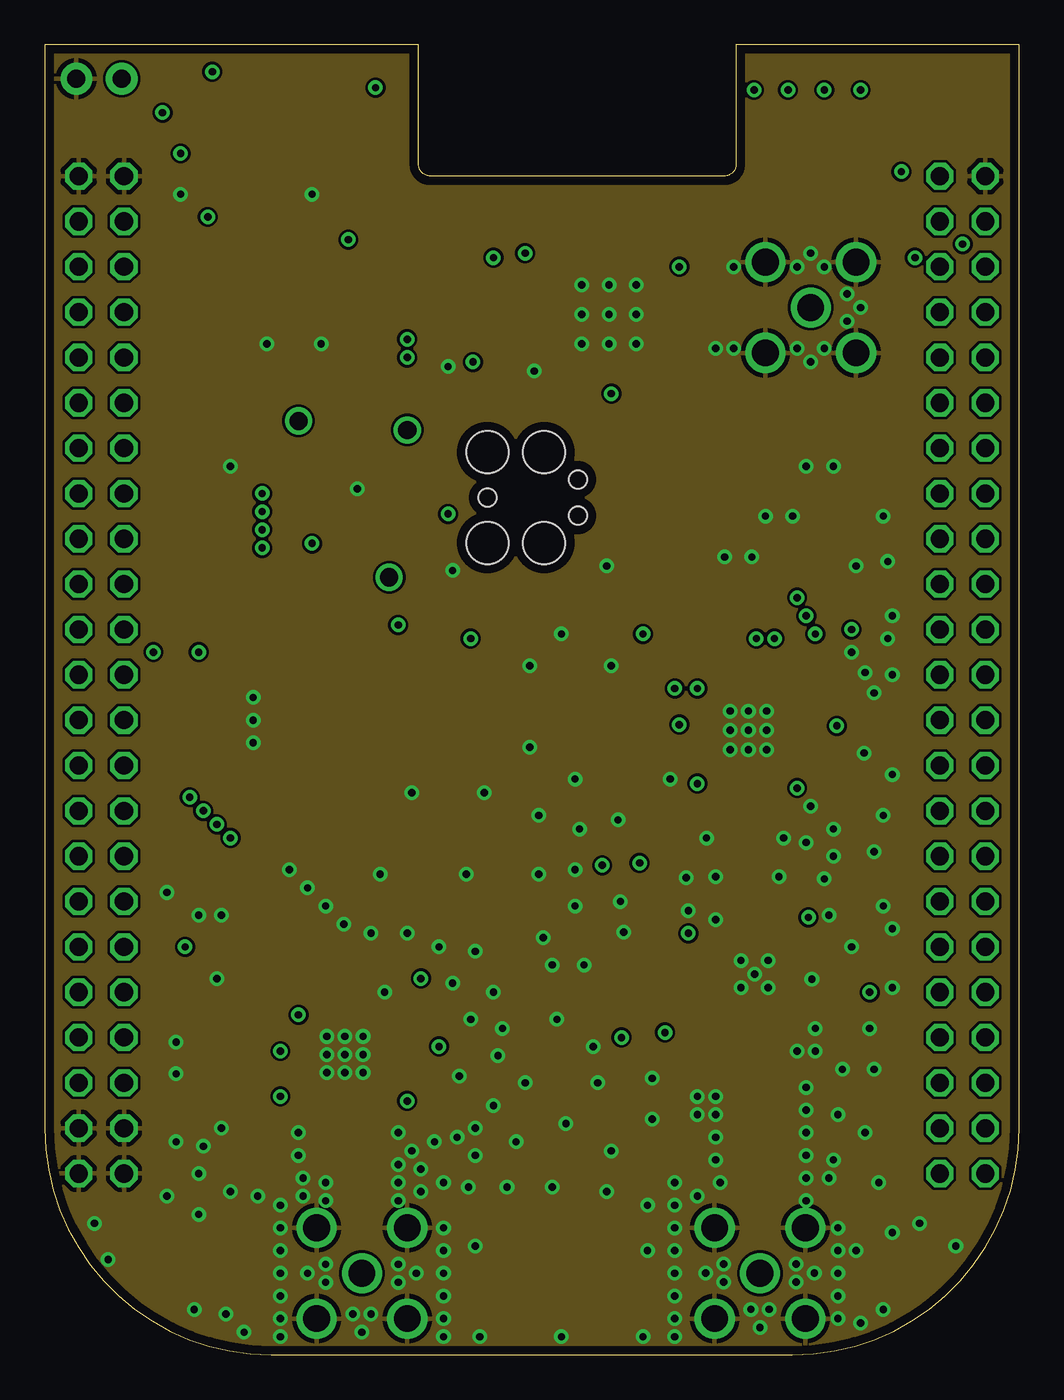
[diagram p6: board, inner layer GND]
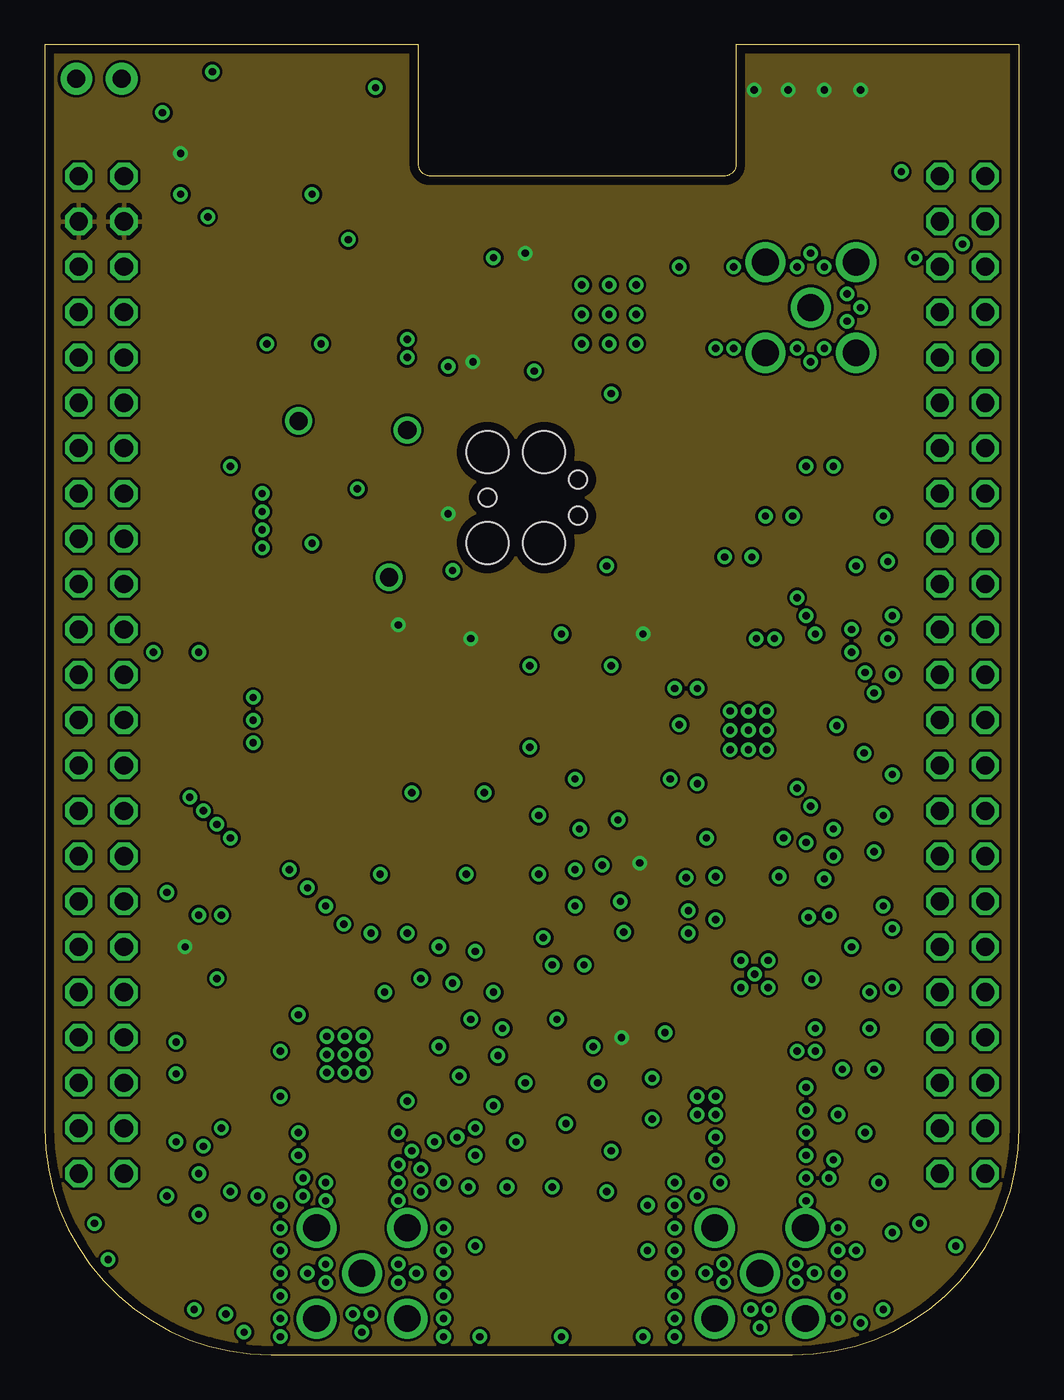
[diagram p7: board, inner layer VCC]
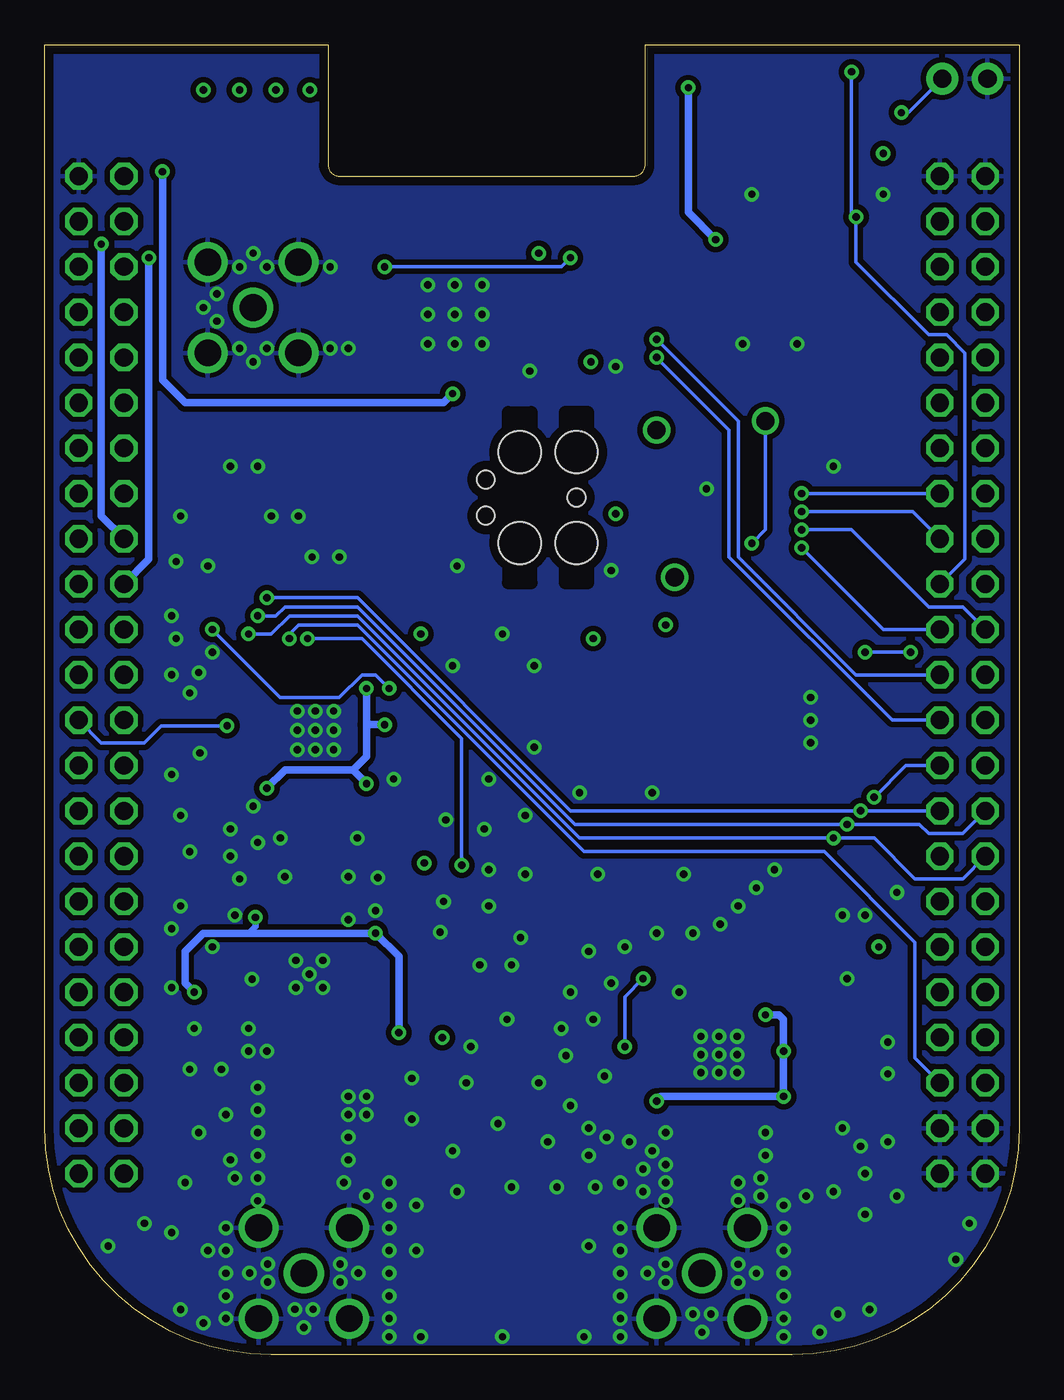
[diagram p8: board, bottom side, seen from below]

Size 54.61 x 73.41 mm. Coordinates in mm from the lower left corner, seen from the top.
Outline: 0,73.41 0,12.7 arc90 12.7,0 41.91,0 arc90 54.61,12.7 54.61,73.41 38.73,73.41 38.73,66.67 arc-90 38.1,66.04 21.59,66.04 arc-90 20.95,66.67 20.95,73.41 0,73.41
Copper layers (1+2*15+16): Top 0.0178mm / dielectric 12mil / GND 0.0356mm / dielectric 28mil / VCC 0.0356mm / dielectric 12mil / Bottom 0.0178mm
Design rules "sunstone-4lyr_v1.0.0.3 *": minimum track width 6mil, minimum drill 8mil, track to track 6mil, track to pad 6mil, pad to pad 6mil, via to via 6mil, smd to smd 6mil, copper to edge 20mil, drill to drill 16mil, minimum pad ring 8mil, minimum via ring 8mil, stop-mask expansion 3mil, vias tented up to drill 25mil, thermal gap 10mil

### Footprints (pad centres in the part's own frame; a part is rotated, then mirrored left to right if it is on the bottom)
MOLEX_WM5544-ND = drill 1.499: GND1 0,5.08; GND2 5.08,5.08; GND3 0,0; GND4 5.08,0; SIGNAL 2.54,2.54
2450BM = smd 0.35 x 1: 1 0.65,0.9; 2 0,0.9; 3 -0.65,0.9; 4 -0.65,-0.9; 5 0,-0.9; 6 0.65,-0.9
BAL-NRF01D3 = smd 0.22 x 0.22: ANT1 -0.537,-0.25; ANT2 -0.537,0.25; GND 0.069,0.25; SE 0.537,0; VCC 0.069,-0.25
0402_CAP = smd 0.536 x 0.546: 1 -0.433,0; 2 0.433,0
C0402 = smd 0.536 x 0.546: 1 -0.433,0; 2 0.433,0
C0603 = smd 1.1 x 1: 1 -0.85,0; 2 0.85,0
LED-0603 = smd 1 x 1: A 0,-0.877; C 0,0.877
TC2030-IDC = smd 0.787 x 0.787: 1 -1.27,-0.635; 2 -1.27,0.635; 3 0,-0.635; 4 0,0.635; 5 1.27,-0.635; 6 1.27,0.635 | hole 2.375: -2.54,2.54; 0.635,2.54; 0.635,-2.54; -2.54,-2.54 | hole 1.016: -2.54,0; 2.54,1.016; 2.54,-1.016
PTH-JUMPER-2-NO_NO_SILK = drill 1.016 pad 1.778: 1 -1.27,0; 2 1.27,0
0603_CAP = smd 0.7 x 1: 1 -0.65,0; 2 0.65,0
0603 = smd 1.1 x 1: 1 -0.85,0; 2 0.85,0
BBB_HEADERS = drill 1.016 octagon: P8_1 49.53,57.15; P8_2 52.07,57.15; P8_3 49.53,54.61; P8_4 52.07,54.61; P8_5 49.53,52.07; P8_6 52.07,52.07; P8_7 49.53,49.53; P8_8 52.07,49.53; P8_9 49.53,46.99; P8_10 52.07,46.99; P8_11 49.53,44.45; P8_12 52.07,44.45; P8_13 49.53,41.91; P8_14 52.07,41.91; P8_15 49.53,39.37; P8_16 52.07,39.37; P8_17 49.53,36.83; P8_18 52.07,36.83; P8_19 49.53,34.29; P8_20 52.07,34.29; P8_21 49.53,31.75; P8_22 52.07,31.75; P8_23 49.53,29.21; P8_24 52.07,29.21; P8_25 49.53,26.67; P8_26 52.07,26.67; P8_27 49.53,24.13; P8_28 52.07,24.13; P8_29 49.53,21.59; P8_30 52.07,21.59; P8_31 49.53,19.05; P8_32 52.07,19.05; P8_33 49.53,16.51; P8_34 52.07,16.51; P8_35 49.53,13.97; P8_36 52.07,13.97; P8_37 49.53,11.43; P8_38 52.07,11.43; P8_39 49.53,8.89; P8_40 52.07,8.89; P8_41 49.53,6.35; P8_42 52.07,6.35; P8_43 49.53,3.81; P8_44 52.07,3.81; P8_45 49.53,1.27; P8_46 52.07,1.27; P9_1 1.27,57.15; P9_2 3.81,57.15; P9_3 1.27,54.61; P9_4 3.81,54.61; P9_5 1.27,52.07; P9_6 3.81,52.07; P9_7 1.27,49.53; P9_8 3.81,49.53; P9_9 1.27,46.99; P9_10 3.81,46.99; P9_11 1.27,44.45; P9_12 3.81,44.45; P9_13 1.27,41.91; P9_14 3.81,41.91; P9_15 1.27,39.37; P9_16 3.81,39.37; P9_17 1.27,36.83; P9_18 3.81,36.83; P9_19 1.27,34.29; P9_20 3.81,34.29; P9_21 1.27,31.75; P9_22 3.81,31.75; P9_23 1.27,29.21; P9_24 3.81,29.21; P9_25 1.27,26.67; P9_26 3.81,26.67; P9_27 1.27,24.13; P9_28 3.81,24.13; P9_29 1.27,21.59; P9_30 3.81,21.59; P9_31 1.27,19.05; P9_32 3.81,19.05; P9_33 1.27,16.51; P9_34 3.81,16.51; P9_35 1.27,13.97; P9_36 3.81,13.97; P9_37 1.27,11.43; P9_38 3.81,11.43; P9_39 1.27,8.89; P9_40 3.81,8.89; P9_41 1.27,6.35; P9_42 3.81,6.35; P9_43 1.27,3.81; P9_44 3.81,3.81; P9_45 1.27,1.27; P9_46 3.81,1.27
R0402 = smd 0.536 x 0.546: 1 -0.433,0; 2 0.433,0
0603-RES = smd 0.7 x 1: 1 -0.65,0; 2 0.65,0
PAD-JUMPER-3-NO_YES_SILK_FULL_BOX = smd 1.168 x 1.6: 1 -1.524,0; 2 0,0; 3 1.524,0
PAD-JUMPER-2-NC_BY_TRACE_YES_SILK = smd 0.635 x 1.27: 1 -0.508,0; 2 0.508,0
TESTPOINT_0.040IN = drill 1.016: TESTPOINT 0,0
TP14SQ = smd 1.4 x 1.4: TP 0,0
S-PVQFN-N28 = smd 1 x 0.28: 1 -2.4,1.5; 2 -2.4,1; 3 -2.4,0.5; 4 -2.4,0; 5 -2.4,-0.5; 6 -2.4,-1; 7 -2.4,-1.5; 15 2.4,-1.5; 16 2.4,-1; 17 2.4,-0.5; 18 2.4,0; 19 2.4,0.5; 20 2.4,1; 21 2.4,1.5 | smd 0.28 x 1: 8 -1.5,-2.4; 9 -1,-2.4; 10 -0.5,-2.4; 11 0,-2.4; 12 0.5,-2.4; 13 1,-2.4; 14 1.5,-2.4; 22 1.5,2.4; 23 1,2.4; 24 0.5,2.4; 25 0,2.4; 26 -0.5,2.4; 27 -1,2.4; 28 -1.5,2.4 | smd 3.15 x 3.15: THERMALPAD 0,0
CAT24C256WI-GT3 = smd 2.2 x 0.6: A0 -2.6,1.91; A1 -2.6,0.65; A2 -2.6,-0.64; SCL 2.6,-0.64; SDA 2.6,-1.91; VCC 2.6,1.91; VSS -2.6,-1.91; WP 2.6,0.64
PVQFN-16 = smd 0.35 x 0.825: 1 -0.975,-2.013; 2 -0.325,-2.013; 3 0.325,-2.013; 4 0.975,-2.013; 9 0.975,2.013; 10 0.325,2.013; 11 -0.325,2.013; 12 -0.975,2.013 | smd 0.825 x 0.35: 5 2.013,-0.975; 6 2.013,-0.325; 7 2.013,0.325; 8 2.013,0.975; 13 -2.013,0.975; 14 -2.013,0.325; 15 -2.013,-0.325; 16 -2.013,-0.975 | smd 2.16 x 2.16: PAD 0,0
TSSOP16 = smd 0.9 x 0.35: 1 -2.875,2.275; 2 -2.875,1.625; 3 -2.875,0.975; 4 -2.875,0.325; 5 -2.875,-0.325; 6 -2.875,-0.975; 7 -2.875,-1.625; 8 -2.875,-2.275; 9 2.875,-2.275; 10 2.875,-1.625; 11 2.875,-0.975; 12 2.875,-0.325; 13 2.875,0.325; 14 2.875,0.975; 15 2.875,1.625; 16 2.875,2.275
QFN-48-6MM = smd 0.8 x 0.25: 1 -3,2.2; 2 -3,1.8; 3 -3,1.4; 4 -3,1; 5 -3,0.6; 6 -3,0.2; 7 -3,-0.2; 8 -3,-0.6; 9 -3,-1; 10 -3,-1.4; 11 -3,-1.8; 12 -3,-2.2; 25 3,-2.2; 26 3,-1.8; 27 3,-1.4; 28 3,-1; 29 3,-0.6; 30 3,-0.2; 31 3,0.2; 32 3,0.6; 33 3,1; 34 3,1.4; 35 3,1.8; 36 3,2.2 | smd 0.25 x 0.8: 13 -2.2,-3; 14 -1.8,-3; 15 -1.4,-3; 16 -1,-3; 17 -0.6,-3; 18 -0.2,-3; 19 0.2,-3; 20 0.6,-3; 21 1,-3; 22 1.4,-3; 23 1.8,-3; 24 2.2,-3; 37 2.2,3; 38 1.8,3; 39 1.4,3; 40 1,3; 41 0.6,3; 42 0.2,3; 43 -0.2,3; 44 -0.6,3; 45 -1,3; 46 -1.4,3; 47 -1.8,3; 48 -2.2,3 | smd 4.6 x 4.6: GND 0,0
NX2520SA = smd 1.2 x 1: 1 -0.85,-0.85; 2 0.85,-0.85; 3 0.85,0.85; 4 -0.85,0.85
TXC-8Y = smd 0.9 x 0.8: 1 -0.7,-0.55; 2 0.7,-0.55; 3 0.7,0.55; 4 -0.7,0.55

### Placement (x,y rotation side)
ANT1  15.24,2.03 0 top
ANT2  37.54,2.03 0 top
ANT3  40.39,56.13 0 top
B1  16.83,11.75 270 top
B2  36.07,58.67 0 top
C1  37.4,59.11 90 top
C2  40.53,15.88 0 top
C3  39.65,11.02 180 top
C4  38.95,29.48 270 top
C5  39.93,29.48 270 top
C6  40.09,14.12 90 top
C7  35.81,63.5 270 top
C8  31.75,63.5 90 top
C9  37.08,16.21 270 top
C10  31.24,31.24 180 top
C11  8.13,19.05 180 top
C12  8.13,14.22 180 top
C13  31.24,35.81 180 top
C14  44.7,19.68 270 top
C15  41.77,25.15 90 top
C16  43.31,22.61 0 top
C17  37.08,61.47 0 top
C18  29.72,63.5 90 top
C19  36.55,57.66 0 top
C20  35.56,55.63 270 top
C21  12.19,13.34 180 top
C22  21.59,13.72 270 top
C23  12.06,21.08 180 top
C24  21.59,19.05 0 top
C25  10.92,66.04 180 top
C26  35.56,30.73 180 top
C27  44.45,31.75 270 top
C28  35.81,38.86 180 top
C29  44.2,37.08 0 top
C30  24.89,55.37 270 top
C31  25.65,60.45 0 top
C32  11.94,11.43 180 top
C33  34.04,28.96 180 top
C34  34.04,24.51 180 top
C35  25.91,55.37 270 top
D1  40.64,70.87 180 top
D2  42.67,70.87 180 top
D3  44.7,70.87 180 top
D4  46.74,70.87 180 top
J1  27.35,48.03 0 top
J2  3.05,71.5 180 top
L1  38.52,27.83 0 top
L2  40.37,27.81 180 top
L3  39.94,26.15 90 top
L4  39.65,12.28 180 top
L5  38.35,17.5 270 top
L6  40.09,17.63 90 top
L7  38.95,26.14 90 top
L8  36.53,18.06 180 top
L9  25.65,58.93 0 top
L10  27.18,59.44 90 top
L11  34.04,26.42 0 top
L12  10.16,22.61 180 top
L13  35.31,41.4 180 top
P9/P8  0.64,8.89 0 top
R1  40.64,67.82 90 top
R2  42.67,67.82 90 top
R3  44.7,67.82 90 top
R4  46.74,67.82 90 top
R5  33.02,22.61 180 top
R6  33.02,20.83 180 top
R7  45.49,21.67 180 top
R8  13.46,66.04 180 top
R9  13.46,64.14 180 top
R10  13.46,62.23 180 top
R11  10.92,62.23 0 top
R12  10.92,64.14 0 top
R13  7.87,69.09 90 top
R14  23.62,37.85 0 top
R15  22.35,39.12 0 top
R16  22.35,41.15 0 top
R17  34.17,53.38 0 top
R18  21.59,15.43 180 top
R19  44.2,33.78 180 top
R20  33.02,19.05 180 top
R21  18.92,21.34 180 top
R22  43.94,42.16 180 top
SJ1  18.16,65.91 0 top
SJ2  18.29,33.27 180 top
TP0  14.22,52.32 0 top
TP1  19.3,43.56 0 top
TP2  20.32,51.82 0 top
TP3  14.48,33.27 0 top
U1  16.83,16.83 270 top
U2  39.43,35 270 top
U3  13.72,70.36 180 top
U4  39.78,21.34 180 top
U5  17.02,37.59 0 top
U6  31.54,58.29 0 top
U$2  [UMICH_SOLID_200MIL]  5.08,3.05 0 top
X1  9.65,16.64 90 top
X2  32.73,33.53 90 top
X3  33.53,63.5 180 top

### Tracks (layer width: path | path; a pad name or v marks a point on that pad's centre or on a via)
5V
  Top 0.406: P9/P8.P9_7 P9/P8.P9_8
!RESET0  (via drill 0.41)
  Top 0.203: v22.1,17.27 21.65,16.83 U1.25 | v21.08,21.08 21.08,21.84 20.07,22.86 16.51,22.86 11.43,27.94 11.43,29.46 7.87,33.02 7.87,49.91 P9/P8.P9_12
  Bottom 0.203: v22.1,17.27 22.1,20.07 v21.08,21.08
!RESET1  (via drill 0.41)
  Top 0.203: U2.25 44.15,35 v44.39,35.24
  Bottom 0.203: v44.39,35.24 48.07,35.24 49.02,34.29 51.44,34.29 P9/P8.P8_26
!RESET2
  Top 0.203: U6.8 8.42,57.69 5.33,54.61 3.17,54.61 P9/P8.P9_11
AVDD  (via drill 0.41)
  Top 0.203: C17.1 36.07,61.47 v35.56,60.96 35.09,60.49 | 35.05,60.45 35.05,60.2 34.95,60.09 U6.35 | 35.09,60.49 U6.36 35.01,60.49 35.05,60.45 | 35.05,60.45 35.09,60.49 | v25.15,61.47 25.15,60.53 C31.1 L9.1
  Bottom 0.203: v35.56,60.96 25.65,60.96 v25.15,61.47
BIRQ  (via drill 0.41)
  Top 0.203: v12.19,48.26 12.7,48.26 19.3,54.86 20.83,54.86 22.46,56.49 U6.11
  Bottom 0.203: v12.19,48.26 P9/P8.P9_16
CCA0
  Top 0.203: U1.6 15.83,20.49 6.86,29.46 6.86,45.47 5.33,46.99 3.17,46.99 P9/P8.P9_15
CCA1
  Top 0.203: U2.6 38.43,40.72 47.24,49.53 51.44,49.53 P9/P8.P8_14
DCC
  Top 0.203: U6.2 L10.2
EN
  Top 0.203: U2.10 36.44,35.5 35.88,36.07 35.31,36.07 34.29,37.08 30.23,37.08 28.7,35.56 28.7,24.5 32.37,20.83 R6.2
FIFO0
  Top 0.203: U1.9 13.67,17.83 11.43,20.07 8.64,20.07 5.84,22.86 5.84,30.99 5.08,31.75 3.17,31.75 P9/P8.P9_27
FIFO1  (via drill 0.41)
  Top 0.203: U2.9 36.58,36 35.31,37.27 v35.31,37.34 | P9/P8.P8_16 51.44,46.99 49.53,46.99 48.77,46.23 48.77,44.2 v45.21,40.64
  Bottom 0.203: v35.31,37.34 36.07,38.1 36.83,38.1 38.1,36.83 41.4,36.83 v45.21,40.64
FIFOP0
  Top 0.203: U1.7 15.33,20.49 6.35,29.46 6.35,36.07 5.59,36.83 3.17,36.83 P9/P8.P9_23
FIFOP1
  Top 0.203: P9/P8.P8_13 47.75,50.8 37.93,40.98 U2.7
GND  (via drill 0.41)
  Top 0.203: 34.65,59.29 U6.33 35.04,59.29 35.18,59.44 35.18,59.56 35.05,59.69 U6.34 36.14,59.69 37.25,59.69 C1.2 37.4,60.52 37.59,60.71 38.35,60.71 v38.61,60.96 | C19.2 36.99,56.99 v37.59,56.39 | U6.13 27.61,55.29 v27.43,55.12 | J1.5 28.62,47.07 v31.5,44.2 | R21.1 19.3,21.34 19.3,20.57 v19.05,20.32
  Top 0.305: 36.13,59.29 36.13,58.93 B2.GND 36.14,59.69
  Top 0.356: B1.2 19.62,11.75 19.81,11.94 v19.81,12.45
  Top 0.406: U4.PAD 39.78,22.1 | R19.1 45.85,33.78 v45.91,33.72
  other vias: 23.24,15.62 42.99,21.04 9.65,21.08 9.91,24.64 6.86,25.91 8.64,24.64 9.91,12.7 8.89,11.68 7.37,11.94 7.37,15.75 7.37,17.53 10.41,9.14 8.64,10.16 13.21,7.11 15.75,9.65 15.75,8.64 19.81,9.65 19.81,10.67 19.81,8.64 19.81,5.08 19.81,4.06 17.27,2.29 18.29,2.29 15.75,5.08 15.75,4.06 14.73,4.57 17.78,1.27 20.83,4.57 14.22,12.45 14.22,11.18 14.48,8.89 13.21,8.38 13.21,5.84 13.21,4.57 13.21,3.3 13.21,2.03 13.21,1.02 22.35,1.02 22.35,2.03 22.35,3.3 22.35,4.57 22.35,5.84 22.35,7.11 14.48,9.91 21.08,9.14 22.35,9.65 21.84,11.94 21.08,10.41 20.57,11.43 8.38,2.54 3.56,5.33 2.79,7.37 11.18,1.27 13.72,27.18 14.73,26.16 15.75,25.15 16.76,24.13 18.29,23.62 20.32,23.62 22.1,22.86 22.86,20.83 23.88,18.8 25.4,16.76 25.15,13.97 24.13,12.7 24.13,22.61 25.15,20.32 25.65,18.29 26.92,15.24 26.42,11.94 24.13,11.18 23.11,12.19 11.94,8.89 6.86,8.89 11.68,35.56 11.68,34.29 31.75,11.43 28.45,9.4 33.78,8.38 23.75,9.4 33.78,5.84 24.38,1.02 33.53,1.02 35.31,1.02 35.31,2.03 35.31,4.57 35.31,5.84 35.31,7.11 35.31,8.38 37.85,9.65 43.94,9.91 38.05,5.09 38.05,4.08 37.03,4.58 39.57,2.55 40.59,2.55 40.08,1.54 42.67,8.64 43.13,4.58 42.11,5.09 42.11,4.08 44.45,4.57 44.45,5.84 44.45,7.11 44.45,3.3 44.45,2.03 35.31,3.3 42.67,9.91 42.67,11.18 42.67,12.45 42.67,13.72 42.67,14.99 42.16,17.02 43.18,17.02 43.18,18.29 37.59,10.92 37.59,12.19 37.59,13.46 37.59,14.48 36.58,14.48 30.99,15.24 34.04,15.49 34.04,13.21 44.2,10.92 44.45,13.46 46.48,16 45.97,12.45 46.74,9.65 49.02,7.37 45.47,5.84 46.99,2.54 51.05,6.1 45.72,1.78 28.96,1.02 31.5,9.14 25.91,9.4 35.31,9.65 36.58,8.89 36.58,13.46 47.5,6.86 30.73,17.27 30.23,21.84 28.7,18.8 28.45,21.84 27.94,23.37 29.72,25.15 29.97,29.46 27.18,34.04 27.69,30.23 24.64,31.5 11.68,36.83 23.62,26.92 27.18,38.61 28.96,40.39 31.75,38.61 43.94,24.64 45.21,22.86 47.5,23.88 46.23,18.29 44.7,16 41.15,26.8 44.2,29.46 42.93,30.73 41.4,28.96 42.67,28.7 43.69,26.67 47.5,20.57 37.59,24.38 36.07,24.89 37.59,26.8 35.94,26.73 35.05,32.26 37.08,28.96 10.41,49.78 22.86,43.94 17.53,48.51 38.1,44.7 40.39,46.99 47.24,44.45 45.47,44.2 41.91,46.99 42.67,49.78 46.99,46.99 47.5,41.4 47.24,40.13 47.5,38.1 46.48,37.08 46.99,30.23 47.5,32.51 46.48,28.19 46.99,25.15 29.21,12.95 16.83,16.83 17.84,16.83 17.84,17.84 16.83,17.84 15.81,17.84 15.81,16.83 15.81,15.81 16.83,15.81 17.84,15.81 39.78,21.34 39.01,22.1 40.54,22.1 39.01,20.57 40.54,20.57 38.42,36.07 39.43,36.07 40.45,36.07 38.42,34.99 39.43,34.99 40.45,34.99 38.42,33.91 39.43,33.91 40.45,33.91 8.64,7.87 10.16,2.29 24.13,6.1 27.69,26.92 29.72,32.26 32.13,29.97 29.72,27.18 45.97,38.23 45.21,39.37 44.2,27.94 32.26,25.4 32.45,23.69 44.2,49.78 39.62,44.7 38.61,56.39 42.16,60.96 43.69,60.96 42.93,61.72 44.96,59.44 44.96,57.91 45.72,58.67 42.16,56.39 43.69,56.39 42.93,55.63 30.1,59.94 31.62,59.94 33.15,59.94 30.1,58.29 31.62,58.29 33.15,58.29 30.1,56.64 31.62,56.64 33.15,56.64 22.61,55.37 12.45,56.64 15.49,56.64 14.99,65.02 7.62,65.02 20.57,31.5 18.8,26.92
  pour Bottom (isolate 0.305): 0,73.41 54.61,73.41 54.61,0 0,0
  pour Top: 54.61,73.41 0,73.41 0,0.02 5.2,0 16,0 16,12.45 19.56,12.45 19.6,0 38.1,0 38.1,9.65 38.86,10.41 38.86,12.83 38.35,13.46 38.35,18.54 37.85,18.54 37.85,32.77 40.89,32.77 40.89,18.8 41.66,18.8 41.66,17.08 41.08,16.51 41.08,15.24 41.15,15.18 41.91,14.48 41.91,0 54.61,0 54.61,56.9 34.8,56.9 34.8,60.45 54.61,60.45
  pour GND: 0,0 54.61,0 54.61,73.41 0,73.41
  pour Top: 19.3,11.94 19.3,3.05 16.26,3.05 16.26,11.94 14.48,11.94 14.48,0 21.08,0 21.08,11.94
  pour Top (no thermals): 36.32,0 36.32,16.51 38.73,16.51 38.73,13.21 39.5,12.83 39.5,10.46 38.57,9.78 38.57,0
  pour Top (no thermals): 41.59,0 41.59,14.67 40.7,15.24 40.7,16.51 41.47,17.08 41.47,18.8 45.47,18.8 45.47,0
  pour Top: 38.1,0 41.91,0 42.11,3.06 38.3,3.06
  pour Top: 36.83,19.05 41.91,19.05 41.91,20.83 36.83,20.83
  pour Top (no thermals): 38.35,22.58 38.35,31.98 36.83,32 36.83,22.61 38.1,22.61
  pour Top (no thermals): 40.55,31.99 40.55,22.59 41.91,22.61 41.91,32
  pour Top: 16,0 16,2.79 19.56,2.79 19.56,0
  pour Top: 54.61,60.71 34.8,60.71 34.8,60.2 44.45,60.2 44.45,57.15 34.8,57.15 34.8,56.64 54.61,56.64
LED0  (via drill 0.41)
  Top 0.406: v48.77,61.47 45.97,64.26 41.4,64.26 40.64,65.02 R1.1
  Bottom 0.406: P9/P8.P8_19 48.77,44.58 v48.77,61.47
LED1  (via drill 0.41)
  Top 0.406: v51.44,62.23 49.15,62.23 46.35,65.02 43.43,65.02 42.67,65.79 R2.1
  Bottom 0.406: v51.44,62.23 51.44,46.99 P9/P8.P8_17
LED2
  Top 0.406: P9/P8.P8_18 53.85,46.86 53.85,64.26 53.34,64.77 48.01,64.77 46.99,65.79 45.21,65.79 44.7,66.29 R3.1
N$1
  Top 0.406: R1.2 D1.C
N$2
  Top 0.406: R2.2 D2.C
N$3
  Top 0.406: R3.2 D3.C
N$5  (via drill 0.41)
  Top 0.203: U1.24 23.95,16.33 24.13,16.51
  Top 0.406: U1.26 20.82,17.33 21.59,18.1 22.54,18.1 24.13,16.51 24.13,15.24 23.11,14.22 v20.32,14.22 | U1.20 17.83,13.67 18.03,13.46 19.56,13.46 v20.32,14.22 | U1.22 19.23,15.32 v20.32,14.22 | U1.16 15.83,13.8 15.49,13.46 12.97,13.46 | v20.32,14.22 21.45,14.22 C22.1 | U1.11 13.4,16.83 v13.21,17.02 | U1.8 14.43,18.85 v14.22,19.05 14.22,20.57 13.72,21.08 C23.1 12.5,21.79 11.94,22.35 11.26,22.35 L12.1 | 12.84,11.48 C32.1 12.62,11.59 C21.1 12.84,13.34 12.97,13.46 | U1.14 14.06,15.33 v13.21,14.48 12.97,14.24 12.97,13.46
  Bottom 0.406: v20.32,14.22 20.07,14.48 v13.21,14.48 v13.21,17.02 13.21,18.8 13.46,19.05 v14.22,19.05
N$7
  Top 0.356: ANT1.SIGNAL 17.78,11.04 B1.1
N$11
  Top 0.203: U1.13 10.54,15.83 X1.1 10.5,15.07 9.65,14.22 C12.1
N$12
  Top 0.203: U1.27 19.93,17.83 C24.1
N$13
  Top 0.203: U1.12 12.37,16.33 11.68,17.02 11.68,18.03 11.18,18.54 9.86,18.54 X1.3 | 8.78,17.51 X1.3 | C11.1 8.56,17.73 X1.3
N$14
  Top 0.203: U1.23 20.76,15.83 R18.2
N$29
  Top 0.406: R8.1 16.51,66.04 SJ1.1 16.64,68.13 U3.A0
N$30
  Top 0.406: U3.A1 15.67,69.6 17.78,69.6 19.68,67.69 SJ1.3 19.68,64.9 18.92,64.14 R9.1
N$31  (via drill 0.41)
  Top 0.203: U3.WP 7.89,69.72 R13.2 7.73,69.6 v6.6,69.6
  Bottom 0.203: v6.6,69.6 6.22,69.6 J2.1
N$32  (via drill 0.41)
  Top 0.406: U3.A2 v18.54,70.99 | R10.1 16.76,62.23 v17.02,62.48
  Bottom 0.406: v17.02,62.48 18.54,64.01 v18.54,70.99
N$36
  Top 0.203: U6.31 35.46,58.49 B2.ANT1
N$37
  Top 0.203: U6.32 35.5,58.89 B2.ANT2
N$38
  Top 0.406: ANT3.SIGNAL B2.SE C1.1
N$39
  Top 0.203: 26.2,58.79 L9.2 26.23,58.79 L10.1
N$40
  Top 0.203: U6.37 33.74,61.68 34.04,61.98 34.54,61.98 35.05,62.48 35.05,63.5 34.8,63.75 | 34.8,63.75 34.52,63.75 X3.1 | 34.8,63.75 34.98,63.93 C7.1
N$41
  Top 0.203: U6.38 33.34,61.91 33.02,62.23 33.02,62.76 X3.3 31.87,62.95 C8.1
N$42
  Top 0.203: U6.39 32.94,61.8 32.51,62.23 30.55,62.23 C18.1
N$43
  Top 0.203: U6.29 35.02,57.69 35.56,57.15 C20.1
N$44
  Top 0.356: U4.4 38.8,25.55 L7.1
N$45
  Top 0.356: U4.2 40.1,25.56 L3.1
N$46
  Top 0.508: C5.2 L2.2 L3.2
N$47
  Top 0.508: C4.2 L1.2 L7.2
N$48
  Top 0.203: L8.1 37.85,18.06 38.26,18.06 | 38.26,18.06 L5.1 | U4.10 39.45,18.85 38.66,18.06 38.26,18.06
N$49  (via drill 0.41)
  Top 0.203: U4.13 44.68,20.36 C14.1 44.73,20.36 46.19,20.36 v46.23,20.32 | v34.76,18.06 L8.2 | U4.16 42.58,22.31 C16.1
  Top 0.406: C16.1 42.87,24.44 v42.8,24.51 42.6,24.71 C15.1 41.77,24.37 U4.1 | v36.07,23.62 35.36,23.62 C34.1 L11.2
  Bottom 0.356: v42.8,24.51 42.8,24 43.18,23.62
  Bottom 0.406: v46.23,20.32 46.74,20.83 46.74,22.61 45.72,23.62 43.18,23.62 v36.07,23.62 34.76,22.31 v34.76,18.06
N$50
  Top 0.203: C9.1 37.08,16.94 37.21,17.07 L5.2
N$51
  Top 0.356: U4.11 L6.2
N$52
  Top 0.356: C3.1 ANT2.SIGNAL
  Top 0.508: C6.1 40.09,12.29 L4.1 C3.1
N$53
  Top 0.508: L6.1 C2.1 C6.2
N$54
  Top 0.203: 44.84,21.66 R7.2 44.79,21.72 41.69,21.72 U4.15
N$55
  Top 0.203: U4.5 33.97,22.31 33.67,22.61 R5.1
N$56
  Top 0.203: U4.6 34.5,21.66 33.67,20.83 R6.1
N$57  (via drill 0.41)
  Top 0.203: U2.24 46.52,34.5 46.74,34.29
  Top 0.406: U2.20 40.43,31.96 40.89,31.5 41.91,31.5 v42.16,31.75 42.67,32.26 | U2.22 42.44,33.5 42.67,33.27 42.67,32.26 | 42.67,32.26 44.38,32.26 C27.1 44.78,32.51 45.97,32.51 46.74,33.27 46.74,34.29 44.96,36.07 43.69,36.07 43.12,35.5 U2.26 | U2.11 35.86,35 v35.56,35.31 | U2.8 37.03,36.88 v36.58,37.34 36.58,38.53 C28.1 36.25,41.31 L13.1 36.46,41.4 | v36.58,32 35.99,31.42 C26.1 35.99,30.06 C33.1 | U2.14 37.03,32.46 v36.58,32 | v36.58,32 37.08,31.5 38.04,31.5 38.43,31.89 U2.16
  Bottom 0.406: v42.16,31.75 41.15,32.77 37.34,32.77 | v36.58,37.34 36.58,35.31 | 36.58,35.31 36.58,33.53 37.34,32.77 | v35.56,35.31 36.58,35.31 | 37.34,32.77 v36.58,32
N$58
  Top 0.203: U2.27 42.46,36 C29.1
N$59
  Top 0.203: U2.13 34.91,34 X2.1 33.58,32.31 32.77,31.5 31.93,31.5 C10.1
N$60
  Top 0.203: U2.12 35.09,34.5 34.29,35.31 32.81,35.31 X2.3 31.88,35.8 C13.1
N$61
  Top 0.203: U2.23 43.54,34 R19.2
N$62
  Top 0.203: R20.1 33.67,19.05 35.63,21.01 U4.7
N$63
  Top 0.406: R4.2 D4.C
N$64  (via drill 0.41)
  Top 0.203: v31.75,53.85 U6.19
  Top 0.406: v48.01,66.29 46.91,67.39 R4.1
  Bottom 0.406: v31.75,53.85 32.26,53.34 46.74,53.34 48.01,54.61 v48.01,66.29
N$65
  Top 0.203: SJ2.1 19.05,33.27 19.81,34.04 19.81,35.24 U5.9
PAEN  (via drill 0.41)
  Top 0.203: v31.24,27.43 31.24,23.73 32.37,22.61 R5.2 | U2.4 39.43,39.69 v39.88,40.13
  Bottom 0.203: v39.88,40.13 36.83,40.13 31.24,34.54 v31.24,27.43
RF_N
  Top 0.254: U1.19 17.33,12.8 B1.3
RF_N2
  Top 0.152: U2.19 C5.1
RF_P
  Top 0.254: U1.17 16.33,12.8 B1.4
RF_P2
  Top 0.152: 38.95,32.6 C4.1
  Top 0.203: U2.17 38.95,32.6
SCL
  Top 0.203: 5.84,60.96 5.84,57.91 5.08,57.15 1.27,57.15 0.76,56.64 0.76,44.32 P9/P8.P9_19 | 5.84,60.96 5.84,70.23 6.61,71 U3.SCL | R11.1 7.11,62.23 5.84,60.96
SDA  (via drill 0.41)
  Top 0.203: U3.SDA 9.78,72.27 v9.4,71.88 | R12.1 9.53,64.14 v9.14,63.75
  Bottom 0.203: v9.4,71.88 9.4,64.01 v9.14,63.75 9.14,61.21 5.08,57.15 4.06,57.15 3.05,56.13 3.05,44.58 P9/P8.P9_20
SFD0
  Top 0.203: U1.5 16.33,20.5 7.37,29.46 7.37,47.88 P9/P8.P9_14
SFD1
  Top 0.203: U2.5 38.93,40.46 46.74,48.26 P9/P8.P8_15
SPI0_CS0  (via drill 0.41)
  Top 0.203: P9/P8.P9_17 1.91,44.83 3.17,43.56 3.17,40.01 3.81,39.37 v6.1,39.37 | v8.64,39.37 12.7,39.37 13.46,38.61 13.97,38.61 | 13.97,38.61 14.1,38.61 | U5.3 13.97,38.57 13.97,38.61
  Bottom 0.203: v6.1,39.37 v8.64,39.37
SPI0_CS0_0  (via drill 0.41)
  Top 0.203: R14.1 23.12,37.92 U5.13 18.98,37.92 17.27,39.62 17.27,43.18 v14.99,45.47
  Bottom 0.203: TP0.TESTPOINT 14.22,46.23 v14.99,45.47
SPI0_CS0_1
  Top 0.203: R15.1 21.37,38.57 U5.14 19.09,38.57 18.54,39.12 18.54,42.8 TP1.TESTPOINT
SPI0_CS0_2
  Top 0.203: 21.34,51.82 22.35,52.83 29.46,52.83 30.94,54.31 U6.17 | U5.15 20.42,39.22 21.34,40.13 21.34,40.64 | TP2.TESTPOINT 21.34,51.82 | 21.34,51.82 21.34,40.64 | R16.1 21.84,41.15 21.34,40.64
SPI0_CS0_3
  Top 0.203: U5.12 18.47,37.27 TP3.TP
SPI0_CS0_SEL0
  Top 0.203: P9/P8.P8_11 43.69,53.34 26.96,36.62 U5.11
SPI0_CS0_SEL1
  Top 0.203: P9/P8.P8_12 51.44,52.07 43.18,52.07 27.08,35.97 U5.10
SPI0_MISO  (via drill 0.41)
  Top 0.203: U6.15 30.14,54.53 29.46,53.85 19.3,53.85 12.95,47.5 12.95,46.99 v12.19,46.23
  Bottom 0.203: P9/P8.P9_21 3.17,41.91 5.08,41.91 9.4,46.23 v12.19,46.23
SPI0_MOSI  (via drill 0.41)
  Top 0.203: U6.14 29.74,54.63 29.46,54.36 19.3,54.36 v12.19,47.24
  Bottom 0.203: P9/P8.P9_18 5.97,47.24 v12.19,47.24
SPI0_SCLK  (via drill 0.41)
  Top 0.203: U6.16 30.54,54.42 29.46,53.34 19.3,53.34 13.46,47.5 13.46,46.48 v12.19,45.21
  Bottom 0.203: P9/P8.P9_22 7.62,40.64 v12.19,45.21
SPI1_CS0  (via drill 0.41)
  Top 0.203: U1.3 17.33,20.01 8.13,29.21 v8.13,31.24
  Bottom 0.203: P9/P8.P9_28 6.35,33.02 v8.13,31.24
SPI1_CS1  (via drill 0.41)
  Top 0.203: U2.3 39.93,39.17 v40.89,40.13
  Bottom 0.203: v40.89,40.13 40.89,40.39 40.39,40.89 37.08,40.89 24.38,28.19 10.92,28.19 5.84,23.11 5.84,16.64 P9/P8.P9_42
SPI1_MISO  (via drill 0.41)
  Top 0.203: U1.1 18.33,21.28 R21.2 17.02,21.34 9.65,28.7 v9.65,29.72 | 43.43,42.02 R22.2 43.43,42.16 v42.67,41.4 42.42,41.15 42.42,39.88 40.93,38.39 U2.1
  Bottom 0.203: P9/P8.P9_29 3.17,29.21 5.08,29.21 5.59,29.72 v9.65,29.72 24.89,29.72 37.08,41.91 41.15,41.91 41.66,41.4 v42.67,41.4
SPI1_MOSI  (via drill 0.41)
  Top 0.203: U1.2 17.83,20.02 8.89,28.96 v8.89,30.48 | U2.2 40.43,38.65 41.66,39.88 41.66,41.91 v42.16,42.42
  Bottom 0.203: P9/P8.P9_30 v8.89,30.48 25.15,30.48 37.08,42.42 v42.16,42.42
SPI1_SCLK  (via drill 0.41)
  Top 0.203: U1.28 19.6,18.33 20.32,19.05 20.32,21.84 19.81,22.35 16.51,22.35 10.41,28.45 v10.41,28.96 | U2.28 41.83,38.53 43.18,39.88 v43.18,40.39
  Bottom 0.203: P9/P8.P9_31 3.17,26.67 5.84,26.67 8.13,28.96 v10.41,28.96 24.64,28.96 37.08,41.4 40.89,41.4 41.91,40.39 v43.18,40.39
SWDCLK
  Top 0.203: U6.24 33.74,53.38 | 33.74,53.38 R17.1 | 33.74,53.38 33.74,50.51 31.27,48.03 27.94,48.03 27.35,48.62 J1.4
SWDIO
  Top 0.203: J1.2 26.42,49 26.42,51.56 27.18,52.32 31.24,52.32 33.34,54.42 U6.23
UARTRX  (via drill 0.41)
  Top 0.203: U6.9 20.72,57.29 v20.32,56.9
  Bottom 0.203: v20.32,56.9 15.75,52.32 15.75,44.7 9.14,38.1 P9/P8.P9_24
UARTTX  (via drill 0.41)
  Top 0.203: U6.10 21.33,56.89 v20.32,55.88
  Bottom 0.203: v20.32,55.88 16.26,51.82 16.26,44.7 7.11,35.56 P9/P8.P9_26
VCC  (via drill 0.41)
  Top 0.203: U3.VCC 7.88,68.45 | R13.1 7.87,67.56 v7.62,67.31 | U6.1 28.15,60.49 v26.92,61.72 | J1.1 25.55,47.4 25.27,47.12 v22.61,47.12 | U6.12 26.2,56.09 C35.1 C30.1 | R14.2 24.05,38.43 23.37,39.12 | 23.37,39.12 R15.2 | R16.2 23.37,41.15 23.88,40.64 v23.88,40.13 23.88,39.62 23.37,39.12 | R20.2 32.32,18.79 v32.32,17.78 | v19.81,40.89 19.89,40.81 U5.16
  Top 0.254: C30.1 24.18,55.8 v24,55.63 | 7.88,68.45 R13.1
  Top 0.406: L12.2 8.13,22.61 v7.87,22.86 | L11.1 33.34,26.42 v33.34,27.56 | L13.2 34.54,41.4 v33.53,40.39 | C25.1 R8.2 R9.2 R10.2 R11.2 | R12.2 C25.1 | D1.A arc45 40.62,71.73 v39.75,70.87 | D2.A arc45 42.44,71.64 v41.66,70.87 | D3.A 44.56,71.74 v43.69,70.87 | D4.A 46.6,71.74 v45.72,70.87 | C25.1 11.36,68.21 U3.VCC
  pour VCC: 0,0 54.61,0 54.61,73.41 0,73.41
VDD
  Top 0.406: P9/P8.P9_6 P9/P8.P9_5
VDD_PA
  Top 0.203: B2.VCC 36.14,57.67 C19.1 35.69,57.66 35.25,58.09 U6.30

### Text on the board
tPlace: EEPROM / WRITE | CS0-0 | nRF-CS | CS0-1 | CS0-3 | GAP | N.Jackson | D | 2015/04/03
tNames: P9 | P8 | GND | 3V3 | 5V | SYS_5V | !RST2 | !RST0 | CSE0 | CSE1 | SFD0 | FIP1 | CCA1 | CCA0 | BIRQ | SFD1 | FIO1 | 0CS0 | 0SI | LD1 | LD2 | SCL | SDA | LD0 | 0SO | 0SCLK | FIP0 | RX | TX | !RST1 | FIO0 | 1CS0 | 1SO | 1SI | 1SCLK
tDocu: CE1 | RXD | TXD | SCL | SDA

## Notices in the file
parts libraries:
SparkFun-LED: Licensing: CC v3.0 Share-Alike You are welcome to use this library for commercial purposes.
SparkFun-Aesthetics: Licensing: Creative Commons ShareAlike 4.0 International - https://creativecommons.org/licenses/by-sa/4.0
